(* Logix 5000 Rung export; software revision 20.05 *)

TYPE ILX34MBSCoilData :   // Coil Data
STRUCT
   Data : BOOL[576];
END_STRUCT
END_TYPE

TYPE ILX34MBSUTIL :
STRUCT
   Node : SINT;
   Function : SINT;
   NodeAddress : INT;
   Count : INT;
   ByteCount : SINT;
   IntAddress : INT;
   CountPlusIntAddr : INT;
   Swap : SINT;
   CmdTimer : TIMER[30];
   CurrentCmd : INT;
   CurrentCmdReset : BOOL;
   CmdDone : BOOL;
   TX_ASSY : SINT[82];
   TXID_Previous : SINT;
   RX_ASSY : SINT[90];
   RXID_Previous : SINT;
   RegBuffer : INT[72];
   CoilBuffer : ILX34MBSCoilData;
   MoveTo : INT;
   MoveFrom : INT;
   MasterTXQuery : BOOL;
   MasterRXResponse : BOOL;
   SlaveQuery : BOOL;
   WaitForResponse : BOOL;
   WaitTimer : TIMER;
   Error : SINT;
   WaitForError : BOOL;
   RegDataControl : CONTROL;
   InArraySize : INT;
   OutArraySize : INT;
   InputDiscreteArraySize : INT;
   OutputDiscreteArraySize : INT;
   InputRegisterArraySize : INT;
   OutputRegisterArraySize : INT;
   InputDiscreteArraySizem1 : INT;
   OutputDiscreteArraySizem1 : INT;
   InputRegisterArraySizem1 : INT;
   OutputRegisterArraySizem1 : INT;
   MaxDiscreteSize : INT;
   MaxRegisterSize : INT;
   Connection : BOOL;
END_STRUCT
END_TYPE

TYPE ILX34MBSData :   // Module Data Storage
STRUCT
   InputBit : BOOL[576];   // Coil/Input Input Data
   InputRegister : INT[500];   // Input/Holding Register Input Data
   OutputBit : BOOL[576];   // Coil/Input Output Data
   OutputRegister : INT[500];   // Input/Holding Register Output Data
END_STRUCT
END_TYPE

TYPE ILX34MBSCmd :   // Commands for module when used as a master.
STRUCT
   Enable : SINT;   // 0=Disable 1=Enable the command: Polling and Trigger allowed. 2=Enable the command: Trigger allowed only.
   Node : INT;   // Node address of the target device on the network (1-255).
   Function : SINT;   // Function code for the command. 1, 2, 3, 4, 5, 6, 15 and 16 allowed for master and slave. 8 allowed for slave only.
   DeviceAddress : DINT;   // Address in remote device associated with the command (0-65535).
   Count : INT;   // Number of points associated with the command.
   InternalAddress : DINT;
   PollInterval : DINT;   // Minimum number of milliseconds between issuance of command (0-2,147,483,647ms).
   Swap : SINT;
   Trigger : BOOL;   // 1=Trigger the message. Can be triggered any time command is enabled.
END_STRUCT
END_TYPE

TYPE ILX34MBSConfig :   // Configure the Module
STRUCT
   Type : SINT;   // 0=Master, 1=Slave
   Slave_ID : SINT;   // Slave ID (1-255)
   Baud_Rate : SINT;   // Baud Rate: 0=19200 2=2400 3=4800 4=9600 5=38400
   Serial_COM : SINT;   // 0=7N2 1=7E1 2=7O1 3=8N1 4=8N2 5=8E1 6=8O1
   Protocol : SINT;   // 0 = ASCII 1 = RTU
   RX_Length : SINT;   // Reserved
   TX_Length : SINT;   // Reserved
   Timeout : DINT;   // Timeout in centiseconds (1/100th of a second)
   Reserved01 : INT;   // Reserved
   Input_Status_Count_1X : INT;   // Input Status (1x) Maximum Address
   Reserved02 : INT;   // Reserved
   Output_Coil_Count_0X : INT;   // Output Coil (0x) Maximum Address
   Reserved03 : INT;   // Reserved
   Input_Register_Count_3X : INT;   // Input Register (3x) Maximum Address
   Reserved04 : INT;   // Reserved
   Holding_Register_Count_4X : INT;   // Holding Register (4x) Maximum Address
   Coldboot : BOOL;   // Reset Module to load configuration changes
END_STRUCT
END_TYPE

TYPE ILX34MBSStatus :   // Module Status
STRUCT
   Module : SINT;   // Module Status 1=Ready for Command 2=Processing Command 3=Waiting for Response 4=Processing Response
   RXCount : DINT;   // Number of messages received.
   TXCount : DINT;   // Number of messages transmitted.
   ErrorCount : DINT;   // Number of errors.
   CmdError : INT[30];
END_STRUCT
END_TYPE

TYPE ILX34MBSModuleDef :   // ILX34MBS Data Type
STRUCT
   DATA : ILX34MBSData;   // Data Storage
   STATUS : ILX34MBSStatus;   // Module Status
   MASTERCMD : ILX34MBSCmd[30];   // Master Commands
   UTIL : ILX34MBSUTIL;
END_STRUCT
END_TYPE

ADD_ON_INSTRUCTION AOI1734MBS_36   (* revision 1.10, vendor ProSoft Technology Inc., ExecutePrescan *)
// Add-On - L1y & 1734 Point I/O modules.
// Revision note:
// V1.7 - Resend command if stale
// V1.8 - Function Code 4 Swap for revision 1.15 or lower
// V1.9 - Built AOI in RSlogix v16
// V1.10 - Removed retranmission logic as it was causing addiitonal slave retransmissions.
// Help:
// Previous Version 1.8 was not able to open up in v16 Rslogix 5000.
// Built it back again to support v16 and up.
VAR_IN_OUT
   Connection_Input : SINT[90]; {required}
   Connection_Output : SINT[82]; {required}
   Connection_Config : INT[198]; {required}
        [5].0   // 0=Master 1=Slave
   MBS : ILX34MBSModuleDef; {required}
END_VAR
VAR
   ByteBuffer : SINT[72];
   ByteMoveBuffer : SINT[72];
   ByteSwappedRegister : INT[36];
   CurrentCmd : INT;
   CurrentSwapCount : INT;
   IntAddress : INT;
   MJFAULTS : DINT[12];
   ResetCommandTimer : TIMER;
   WordBuffer : INT[36];
   WordByteSwapBuffer : INT[36];
   WordByteSwapMoveBuffer : INT[36];
   WordMoveBuffer : INT[36];
   WordSwappedRegister : INT[36];
END_VAR

ROUTINE Logic   (* ladder *)
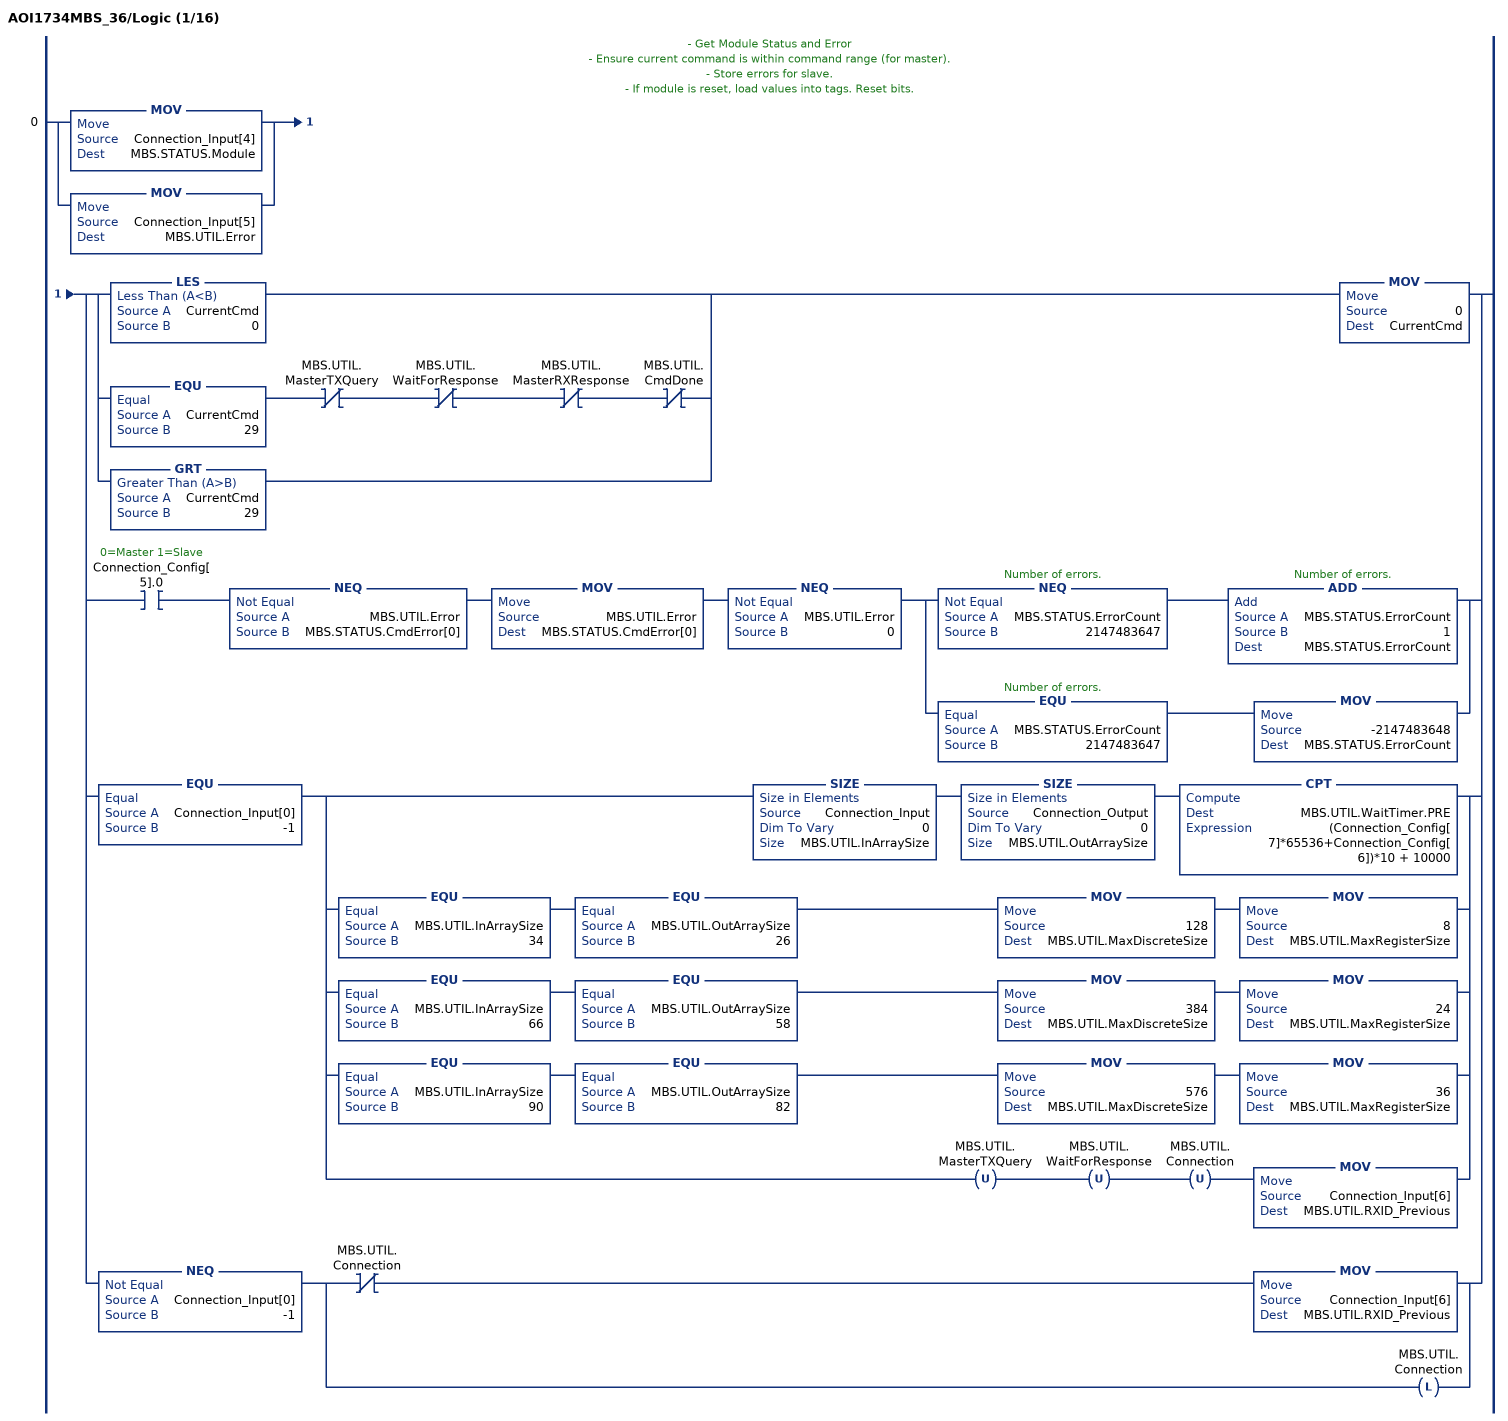
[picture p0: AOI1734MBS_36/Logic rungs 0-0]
   // - Get Module Status and Error
   // - Ensure current command is within command range (for master).
   // - Store errors for slave.
   // - If module is reset, load values into tags. Reset bits.
   0: [MOV(Connection_Input[4],MBS.STATUS.Module) ,MOV(Connection_Input[5],MBS.UTIL.Error) ][[LES(CurrentCmd,0) ,EQU(CurrentCmd,29) XIO(MBS.UTIL.MasterTXQuery) XIO(MBS.UTIL.WaitForResponse) XIO(MBS.UTIL.MasterRXResponse) XIO(MBS.UTIL.CmdDone) ,GRT(CurrentCmd,29) ] MOV(0,CurrentCmd) ,XIC(Connection_Config[5].0) NEQ(MBS.UTIL.Error,MBS.STATUS.CmdError[0]) MOV(MBS.UTIL.Error,MBS.STATUS.CmdError[0]) NEQ(MBS.UTIL.Error,0) [NEQ(MBS.STATUS.ErrorCount,2147483647) ADD(MBS.STATUS.ErrorCount,1,MBS.STATUS.ErrorCount) ,EQU(MBS.STATUS.ErrorCount,2147483647) MOV(-2147483648,MBS.STATUS.ErrorCount) ] ,EQU(Connection_Input[0],-1) [SIZE(Connection_Input,0,MBS.UTIL.InArraySize) SIZE(Connection_Output,0,MBS.UTIL.OutArraySize) CPT(MBS.UTIL.WaitTimer.PRE,(Connection_Config[7]*65536+Connection_Config[6])*10 + 10000) ,EQU(MBS.UTIL.InArraySize,34) EQU(MBS.UTIL.OutArraySize,26) MOV(128,MBS.UTIL.MaxDiscreteSize) MOV(8,MBS.UTIL.MaxRegisterSize) ,EQU(MBS.UTIL.InArraySize,66) EQU(MBS.UTIL.OutArraySize,58) MOV(384,MBS.UTIL.MaxDiscreteSize) MOV(24,MBS.UTIL.MaxRegisterSize) ,EQU(MBS.UTIL.InArraySize,90) EQU(MBS.UTIL.OutArraySize,82) MOV(576,MBS.UTIL.MaxDiscreteSize) MOV(36,MBS.UTIL.MaxRegisterSize) ,OTU(MBS.UTIL.MasterTXQuery) OTU(MBS.UTIL.WaitForResponse) OTU(MBS.UTIL.Connection) MOV(Connection_Input[6],MBS.UTIL.RXID_Previous) ] ,NEQ(Connection_Input[0],-1) [XIO(MBS.UTIL.Connection) MOV(Connection_Input[6],MBS.UTIL.RXID_Previous) ,OTL(MBS.UTIL.Connection) ] ];
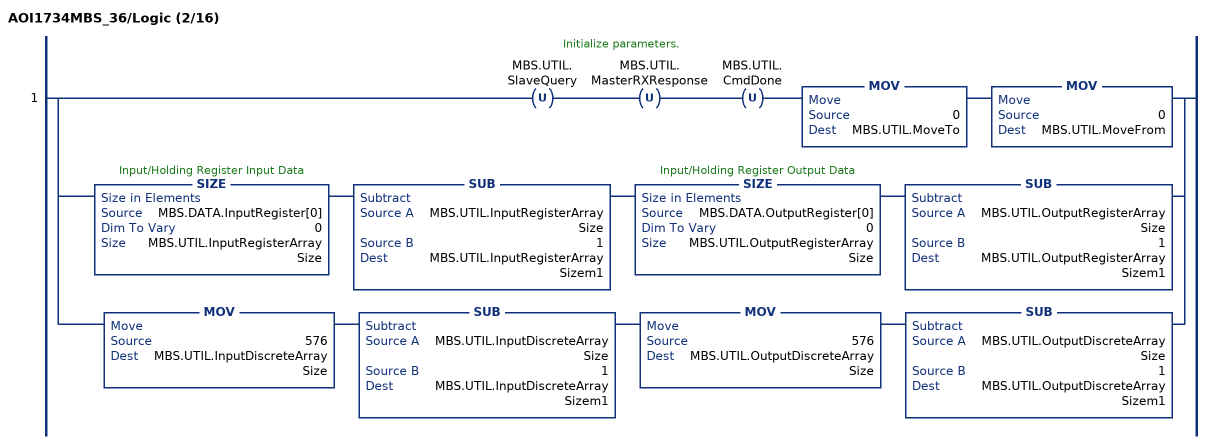
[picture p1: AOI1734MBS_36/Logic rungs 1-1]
   // Initialize parameters.
   1: [OTU(MBS.UTIL.SlaveQuery) OTU(MBS.UTIL.MasterRXResponse) OTU(MBS.UTIL.CmdDone) MOV(0,MBS.UTIL.MoveTo) MOV(0,MBS.UTIL.MoveFrom) ,SIZE(MBS.DATA.InputRegister[0],0,MBS.UTIL.InputRegisterArraySize) SUB(MBS.UTIL.InputRegisterArraySize,1,MBS.UTIL.InputRegisterArraySizem1) SIZE(MBS.DATA.OutputRegister[0],0,MBS.UTIL.OutputRegisterArraySize) SUB(MBS.UTIL.OutputRegisterArraySize,1,MBS.UTIL.OutputRegisterArraySizem1) ,MOV(576,MBS.UTIL.InputDiscreteArraySize) SUB(MBS.UTIL.InputDiscreteArraySize,1,MBS.UTIL.InputDiscreteArraySizem1) MOV(576,MBS.UTIL.OutputDiscreteArraySize) SUB(MBS.UTIL.OutputDiscreteArraySize,1,MBS.UTIL.OutputDiscreteArraySizem1) ];
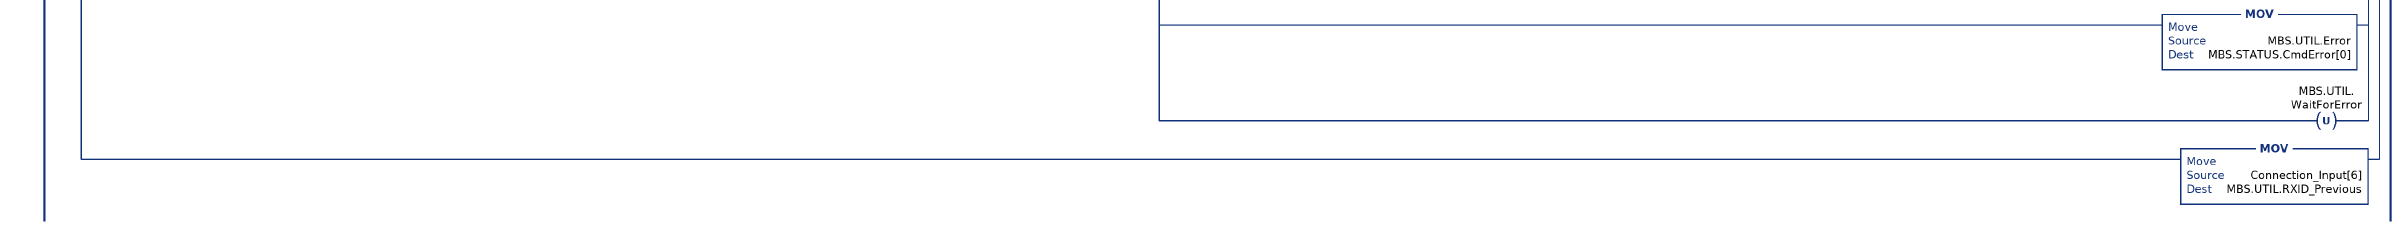
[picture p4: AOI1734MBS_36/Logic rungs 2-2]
   // Receive a message and store into buffer.
   // - If module is a master set response bit.
   // - If module is a slave set query bit (to set up response). Load query info into tags.
   // - If an error occurs in the slave, store type.
   2: NEQ(Connection_Input[6],MBS.UTIL.RXID_Previous)[XIO(Connection_Config[5].0) EQU(Connection_Input[4],1) ,XIC(Connection_Config[5].0) ]COP(Connection_Input[0],MBS.UTIL.RX_ASSY[0],MBS.UTIL.InArraySize)[[MOV(MBS.UTIL.RX_ASSY[4],MBS.STATUS.Module) ,MOV(MBS.UTIL.RX_ASSY[5],MBS.UTIL.Error) ] ,EQU(MBS.UTIL.Error,0) [NEQ(MBS.STATUS.RXCount,2147483647) ADD(1,MBS.STATUS.RXCount,MBS.STATUS.RXCount) ,EQU(MBS.STATUS.RXCount,2147483647) MOV(-2147483648,MBS.STATUS.RXCount) ] ,EQU(MBS.UTIL.Error,0) [XIO(Connection_Config[5].0) EQU(MBS.UTIL.RX_ASSY[8],MBS.UTIL.Function) OTL(MBS.UTIL.MasterRXResponse) ,XIC(Connection_Config[5].0) NEQ(MBS.UTIL.RX_ASSY[8],8) [MOV(MBS.UTIL.RX_ASSY[7],MBS.UTIL.Node) MOV(MBS.UTIL.RX_ASSY[8],MBS.UTIL.Function) COP(MBS.UTIL.RX_ASSY[9],MBS.UTIL.NodeAddress,1) COP(MBS.UTIL.RX_ASSY[11],MBS.UTIL.Count,1) COP(MBS.UTIL.RX_ASSY[9],MBS.UTIL.IntAddress,1) ADD(MBS.UTIL.Count,MBS.UTIL.IntAddress,MBS.UTIL.CountPlusIntAddr) ,[[LIM(1,MBS.UTIL.Function,2) [EQU(MBS.UTIL.Function,1) SUB(MBS.UTIL.IntAddress,Connection_Config[9],MBS.UTIL.IntAddress) ,EQU(MBS.UTIL.Function,2) SUB(MBS.UTIL.IntAddress,Connection_Config[11],MBS.UTIL.IntAddress) ] LIM(0,MBS.UTIL.IntAddress,MBS.UTIL.OutputDiscreteArraySizem1) LIM(1,MBS.UTIL.CountPlusIntAddr,MBS.UTIL.OutputDiscreteArraySize) ,EQU(MBS.UTIL.Function,15) SUB(MBS.UTIL.IntAddress,Connection_Config[9],MBS.UTIL.IntAddress) LIM(0,MBS.UTIL.IntAddress,MBS.UTIL.InputDiscreteArraySizem1) LIM(1,MBS.UTIL.CountPlusIntAddr,MBS.UTIL.InputDiscreteArraySize) ] LIM(1,MBS.UTIL.Count,MBS.UTIL.MaxDiscreteSize) ,[LIM(3,MBS.UTIL.Function,4) [EQU(MBS.UTIL.Function,3) SUB(MBS.UTIL.IntAddress,Connection_Config[15],MBS.UTIL.IntAddress) ,EQU(MBS.UTIL.Function,4) SUB(MBS.UTIL.IntAddress,Connection_Config[13],MBS.UTIL.IntAddress) ] LIM(0,MBS.UTIL.IntAddress,MBS.UTIL.OutputRegisterArraySizem1) LIM(1,MBS.UTIL.CountPlusIntAddr,MBS.UTIL.OutputRegisterArraySize) ,EQU(MBS.UTIL.Function,16) SUB(MBS.UTIL.IntAddress,Connection_Config[15],MBS.UTIL.IntAddress) LIM(0,MBS.UTIL.IntAddress,MBS.UTIL.InputRegisterArraySizem1) LIM(1,MBS.UTIL.CountPlusIntAddr,MBS.UTIL.InputRegisterArraySize) ] LIM(1,MBS.UTIL.Count,MBS.UTIL.MaxRegisterSize) ,EQU(MBS.UTIL.Function,5) LIM(0,MBS.UTIL.IntAddress,MBS.UTIL.InputDiscreteArraySizem1) ,EQU(MBS.UTIL.Function,6) SUB(MBS.UTIL.IntAddress,Connection_Config[15],MBS.UTIL.IntAddress) LIM(0,MBS.UTIL.IntAddress,MBS.UTIL.InputRegisterArraySizem1) ] [OTL(MBS.UTIL.SlaveQuery) ,MOV(MBS.UTIL.IntAddress,IntAddress) ] ] ] ,XIC(Connection_Config[5].0) NEQ(MBS.UTIL.Error,1) NEQ(MBS.UTIL.Error,2) NEQ(MBS.UTIL.Error,3) MOV(MBS.UTIL.Error,MBS.STATUS.CmdError[0]) NEQ(MBS.UTIL.Error,0) [NEQ(MBS.STATUS.ErrorCount,2147483647) ADD(MBS.STATUS.ErrorCount,1,MBS.STATUS.ErrorCount) ,EQU(MBS.STATUS.ErrorCount,2147483647) MOV(-2147483648,MBS.STATUS.ErrorCount) ,MOV(MBS.UTIL.Error,MBS.STATUS.CmdError[0]) ,OTU(MBS.UTIL.WaitForError) ] ,MOV(Connection_Input[6],MBS.UTIL.RXID_Previous) ];
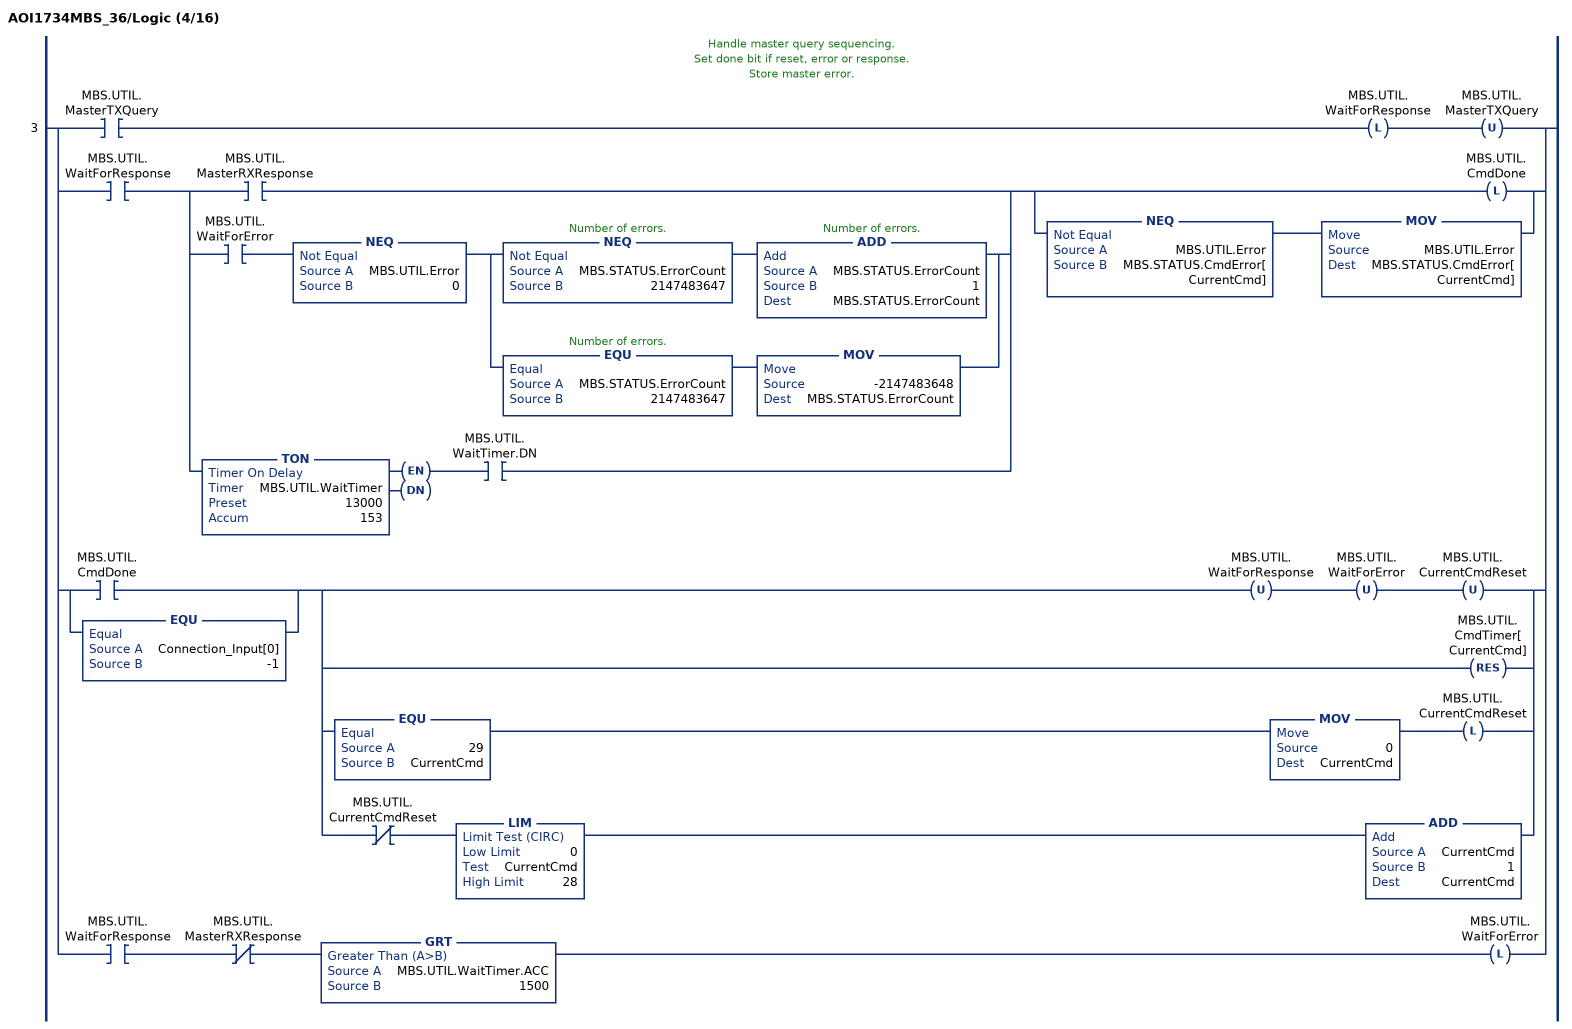
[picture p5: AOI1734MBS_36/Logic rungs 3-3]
   // Handle master query sequencing.
   // Set done bit if reset, error or response.
   // Store master error.
   3: [XIC(MBS.UTIL.MasterTXQuery) OTL(MBS.UTIL.WaitForResponse) OTU(MBS.UTIL.MasterTXQuery) ,XIC(MBS.UTIL.WaitForResponse) [XIC(MBS.UTIL.MasterRXResponse) ,XIC(MBS.UTIL.WaitForError) NEQ(MBS.UTIL.Error,0) [NEQ(MBS.STATUS.ErrorCount,2147483647) ADD(MBS.STATUS.ErrorCount,1,MBS.STATUS.ErrorCount) ,EQU(MBS.STATUS.ErrorCount,2147483647) MOV(-2147483648,MBS.STATUS.ErrorCount) ] ,TON(MBS.UTIL.WaitTimer,13000,153) XIC(MBS.UTIL.WaitTimer.DN) ] [OTL(MBS.UTIL.CmdDone) ,NEQ(MBS.UTIL.Error,MBS.STATUS.CmdError[CurrentCmd]) MOV(MBS.UTIL.Error,MBS.STATUS.CmdError[CurrentCmd]) ] ,[XIC(MBS.UTIL.CmdDone) ,EQU(Connection_Input[0],-1) ] [OTU(MBS.UTIL.WaitForResponse) OTU(MBS.UTIL.WaitForError) OTU(MBS.UTIL.CurrentCmdReset) ,RES(MBS.UTIL.CmdTimer[CurrentCmd]) ,EQU(29,CurrentCmd) MOV(0,CurrentCmd) OTL(MBS.UTIL.CurrentCmdReset) ,XIO(MBS.UTIL.CurrentCmdReset) LIM(0,CurrentCmd,28) ADD(CurrentCmd,1,CurrentCmd) ] ,XIC(MBS.UTIL.WaitForResponse) XIO(MBS.UTIL.MasterRXResponse) GRT(MBS.UTIL.WaitTimer.ACC,1500) OTL(MBS.UTIL.WaitForError) ];
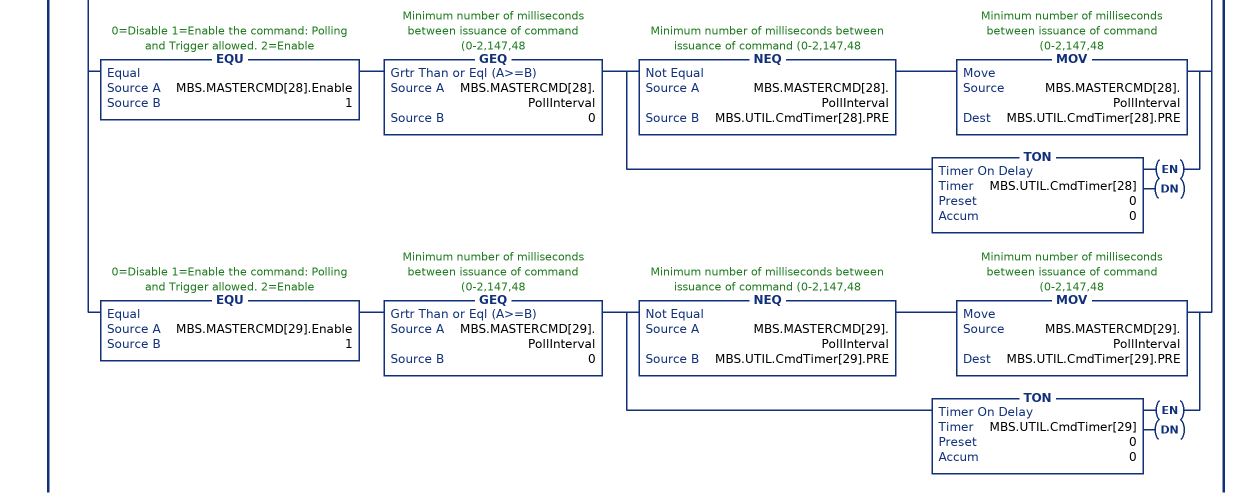
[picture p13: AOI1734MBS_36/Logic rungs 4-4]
   // Master command timers (from Poll Interval).
   // A timer runs only when command enabled = 1. Timers are reset in rung above.
   4: XIO(Connection_Config[5].0)[EQU(MBS.MASTERCMD[0].Enable,1) GEQ(MBS.MASTERCMD[0].PollInterval,0) [NEQ(MBS.MASTERCMD[0].PollInterval,MBS.UTIL.CmdTimer[0].PRE) MOV(MBS.MASTERCMD[0].PollInterval,MBS.UTIL.CmdTimer[0].PRE) ,TON(MBS.UTIL.CmdTimer[0],0,0) ] ,EQU(MBS.MASTERCMD[1].Enable,1) GEQ(MBS.MASTERCMD[1].PollInterval,0) [NEQ(MBS.MASTERCMD[1].PollInterval,MBS.UTIL.CmdTimer[1].PRE) MOV(MBS.MASTERCMD[1].PollInterval,MBS.UTIL.CmdTimer[1].PRE) ,TON(MBS.UTIL.CmdTimer[1],0,0) ] ,EQU(MBS.MASTERCMD[2].Enable,1) GEQ(MBS.MASTERCMD[2].PollInterval,0) [NEQ(MBS.MASTERCMD[2].PollInterval,MBS.UTIL.CmdTimer[2].PRE) MOV(MBS.MASTERCMD[2].PollInterval,MBS.UTIL.CmdTimer[2].PRE) ,TON(MBS.UTIL.CmdTimer[2],0,0) ] ,EQU(MBS.MASTERCMD[3].Enable,1) GEQ(MBS.MASTERCMD[3].PollInterval,0) [NEQ(MBS.MASTERCMD[3].PollInterval,MBS.UTIL.CmdTimer[3].PRE) MOV(MBS.MASTERCMD[3].PollInterval,MBS.UTIL.CmdTimer[3].PRE) ,TON(MBS.UTIL.CmdTimer[3],0,0) ] ,EQU(MBS.MASTERCMD[4].Enable,1) GEQ(MBS.MASTERCMD[4].PollInterval,0) [NEQ(MBS.MASTERCMD[4].PollInterval,MBS.UTIL.CmdTimer[4].PRE) MOV(MBS.MASTERCMD[4].PollInterval,MBS.UTIL.CmdTimer[4].PRE) ,TON(MBS.UTIL.CmdTimer[4],0,0) ] ,EQU(MBS.MASTERCMD[5].Enable,1) GEQ(MBS.MASTERCMD[5].PollInterval,0) [NEQ(MBS.MASTERCMD[5].PollInterval,MBS.UTIL.CmdTimer[5].PRE) MOV(MBS.MASTERCMD[5].PollInterval,MBS.UTIL.CmdTimer[5].PRE) ,TON(MBS.UTIL.CmdTimer[5],0,3) ] ,EQU(MBS.MASTERCMD[6].Enable,1) GEQ(MBS.MASTERCMD[6].PollInterval,0) [NEQ(MBS.MASTERCMD[6].PollInterval,MBS.UTIL.CmdTimer[6].PRE) MOV(MBS.MASTERCMD[6].PollInterval,MBS.UTIL.CmdTimer[6].PRE) ,TON(MBS.UTIL.CmdTimer[6],0,4) ] ,EQU(MBS.MASTERCMD[7].Enable,1) GEQ(MBS.MASTERCMD[7].PollInterval,0) [NEQ(MBS.MASTERCMD[7].PollInterval,MBS.UTIL.CmdTimer[7].PRE) MOV(MBS.MASTERCMD[7].PollInterval,MBS.UTIL.CmdTimer[7].PRE) ,TON(MBS.UTIL.CmdTimer[7],0,0) ] ,EQU(MBS.MASTERCMD[8].Enable,1) GEQ(MBS.MASTERCMD[8].PollInterval,0) [NEQ(MBS.MASTERCMD[8].PollInterval,MBS.UTIL.CmdTimer[8].PRE) MOV(MBS.MASTERCMD[8].PollInterval,MBS.UTIL.CmdTimer[8].PRE) ,TON(MBS.UTIL.CmdTimer[8],0,0) ] ,EQU(MBS.MASTERCMD[9].Enable,1) GEQ(MBS.MASTERCMD[9].PollInterval,0) [NEQ(MBS.MASTERCMD[9].PollInterval,MBS.UTIL.CmdTimer[9].PRE) MOV(MBS.MASTERCMD[9].PollInterval,MBS.UTIL.CmdTimer[9].PRE) ,TON(MBS.UTIL.CmdTimer[9],0,0) ] ,EQU(MBS.MASTERCMD[10].Enable,1) GEQ(MBS.MASTERCMD[10].PollInterval,0) [NEQ(MBS.MASTERCMD[10].PollInterval,MBS.UTIL.CmdTimer[10].PRE) MOV(MBS.MASTERCMD[10].PollInterval,MBS.UTIL.CmdTimer[10].PRE) ,TON(MBS.UTIL.CmdTimer[10],0,0) ] ,EQU(MBS.MASTERCMD[11].Enable,1) GEQ(MBS.MASTERCMD[11].PollInterval,0) [NEQ(MBS.MASTERCMD[11].PollInterval,MBS.UTIL.CmdTimer[11].PRE) MOV(MBS.MASTERCMD[11].PollInterval,MBS.UTIL.CmdTimer[11].PRE) ,TON(MBS.UTIL.CmdTimer[11],0,0) ] ,EQU(MBS.MASTERCMD[12].Enable,1) GEQ(MBS.MASTERCMD[12].PollInterval,0) [NEQ(MBS.MASTERCMD[12].PollInterval,MBS.UTIL.CmdTimer[12].PRE) MOV(MBS.MASTERCMD[12].PollInterval,MBS.UTIL.CmdTimer[12].PRE) ,TON(MBS.UTIL.CmdTimer[12],0,0) ] ,EQU(MBS.MASTERCMD[13].Enable,1) GEQ(MBS.MASTERCMD[13].PollInterval,0) [NEQ(MBS.MASTERCMD[13].PollInterval,MBS.UTIL.CmdTimer[13].PRE) MOV(MBS.MASTERCMD[13].PollInterval,MBS.UTIL.CmdTimer[13].PRE) ,TON(MBS.UTIL.CmdTimer[13],0,0) ] ,EQU(MBS.MASTERCMD[14].Enable,1) GEQ(MBS.MASTERCMD[14].PollInterval,0) [NEQ(MBS.MASTERCMD[14].PollInterval,MBS.UTIL.CmdTimer[14].PRE) MOV(MBS.MASTERCMD[14].PollInterval,MBS.UTIL.CmdTimer[14].PRE) ,TON(MBS.UTIL.CmdTimer[14],0,0) ] ,EQU(MBS.MASTERCMD[15].Enable,1) GEQ(MBS.MASTERCMD[15].PollInterval,0) [NEQ(MBS.MASTERCMD[15].PollInterval,MBS.UTIL.CmdTimer[15].PRE) MOV(MBS.MASTERCMD[15].PollInterval,MBS.UTIL.CmdTimer[15].PRE) ,TON(MBS.UTIL.CmdTimer[15],0,0) ] ,EQU(MBS.MASTERCMD[16].Enable,1) GEQ(MBS.MASTERCMD[16].PollInterval,0) [NEQ(MBS.MASTERCMD[16].PollInterval,MBS.UTIL.CmdTimer[16].PRE) MOV(MBS.MASTERCMD[16].PollInterval,MBS.UTIL.CmdTimer[16].PRE) ,TON(MBS.UTIL.CmdTimer[16],0,0) ] ,EQU(MBS.MASTERCMD[17].Enable,1) GEQ(MBS.MASTERCMD[17].PollInterval,0) [NEQ(MBS.MASTERCMD[17].PollInterval,MBS.UTIL.CmdTimer[17].PRE) MOV(MBS.MASTERCMD[17].PollInterval,MBS.UTIL.CmdTimer[17].PRE) ,TON(MBS.UTIL.CmdTimer[17],0,0) ] ,EQU(MBS.MASTERCMD[18].Enable,1) GEQ(MBS.MASTERCMD[18].PollInterval,0) [NEQ(MBS.MASTERCMD[18].PollInterval,MBS.UTIL.CmdTimer[18].PRE) MOV(MBS.MASTERCMD[18].PollInterval,MBS.UTIL.CmdTimer[18].PRE) ,TON(MBS.UTIL.CmdTimer[18],2000,0) ] ,EQU(MBS.MASTERCMD[19].Enable,1) GEQ(MBS.MASTERCMD[19].PollInterval,0) [NEQ(MBS.MASTERCMD[19].PollInterval,MBS.UTIL.CmdTimer[19].PRE) MOV(MBS.MASTERCMD[19].PollInterval,MBS.UTIL.CmdTimer[19].PRE) ,TON(MBS.UTIL.CmdTimer[19],0,0) ] ,EQU(MBS.MASTERCMD[20].Enable,1) GEQ(MBS.MASTERCMD[20].PollInterval,0) [NEQ(MBS.MASTERCMD[20].PollInterval,MBS.UTIL.CmdTimer[20].PRE) MOV(MBS.MASTERCMD[20].PollInterval,MBS.UTIL.CmdTimer[20].PRE) ,TON(MBS.UTIL.CmdTimer[20],0,0) ] ,EQU(MBS.MASTERCMD[21].Enable,1) GEQ(MBS.MASTERCMD[21].PollInterval,0) [NEQ(MBS.MASTERCMD[21].PollInterval,MBS.UTIL.CmdTimer[21].PRE) MOV(MBS.MASTERCMD[21].PollInterval,MBS.UTIL.CmdTimer[21].PRE) ,TON(MBS.UTIL.CmdTimer[21],0,0) ] ,EQU(MBS.MASTERCMD[22].Enable,1) GEQ(MBS.MASTERCMD[22].PollInterval,0) [NEQ(MBS.MASTERCMD[22].PollInterval,MBS.UTIL.CmdTimer[22].PRE) MOV(MBS.MASTERCMD[22].PollInterval,MBS.UTIL.CmdTimer[22].PRE) ,TON(MBS.UTIL.CmdTimer[22],0,0) ] ,EQU(MBS.MASTERCMD[23].Enable,1) GEQ(MBS.MASTERCMD[23].PollInterval,0) [NEQ(MBS.MASTERCMD[23].PollInterval,MBS.UTIL.CmdTimer[23].PRE) MOV(MBS.MASTERCMD[23].PollInterval,MBS.UTIL.CmdTimer[23].PRE) ,TON(MBS.UTIL.CmdTimer[23],0,0) ] ,EQU(MBS.MASTERCMD[24].Enable,1) GEQ(MBS.MASTERCMD[24].PollInterval,0) [NEQ(MBS.MASTERCMD[24].PollInterval,MBS.UTIL.CmdTimer[24].PRE) MOV(MBS.MASTERCMD[24].PollInterval,MBS.UTIL.CmdTimer[24].PRE) ,TON(MBS.UTIL.CmdTimer[24],0,0) ] ,EQU(MBS.MASTERCMD[25].Enable,1) GEQ(MBS.MASTERCMD[25].PollInterval,0) [NEQ(MBS.MASTERCMD[25].PollInterval,MBS.UTIL.CmdTimer[25].PRE) MOV(MBS.MASTERCMD[25].PollInterval,MBS.UTIL.CmdTimer[25].PRE) ,TON(MBS.UTIL.CmdTimer[25],0,0) ] ,EQU(MBS.MASTERCMD[26].Enable,1) GEQ(MBS.MASTERCMD[26].PollInterval,0) [NEQ(MBS.MASTERCMD[26].PollInterval,MBS.UTIL.CmdTimer[26].PRE) MOV(MBS.MASTERCMD[26].PollInterval,MBS.UTIL.CmdTimer[26].PRE) ,TON(MBS.UTIL.CmdTimer[26],0,0) ] ,EQU(MBS.MASTERCMD[27].Enable,1) GEQ(MBS.MASTERCMD[27].PollInterval,0) [NEQ(MBS.MASTERCMD[27].PollInterval,MBS.UTIL.CmdTimer[27].PRE) MOV(MBS.MASTERCMD[27].PollInterval,MBS.UTIL.CmdTimer[27].PRE) ,TON(MBS.UTIL.CmdTimer[27],0,0) ] ,EQU(MBS.MASTERCMD[28].Enable,1) GEQ(MBS.MASTERCMD[28].PollInterval,0) [NEQ(MBS.MASTERCMD[28].PollInterval,MBS.UTIL.CmdTimer[28].PRE) MOV(MBS.MASTERCMD[28].PollInterval,MBS.UTIL.CmdTimer[28].PRE) ,TON(MBS.UTIL.CmdTimer[28],0,0) ] ,EQU(MBS.MASTERCMD[29].Enable,1) GEQ(MBS.MASTERCMD[29].PollInterval,0) [NEQ(MBS.MASTERCMD[29].PollInterval,MBS.UTIL.CmdTimer[29].PRE) MOV(MBS.MASTERCMD[29].PollInterval,MBS.UTIL.CmdTimer[29].PRE) ,TON(MBS.UTIL.CmdTimer[29],0,0) ] ];
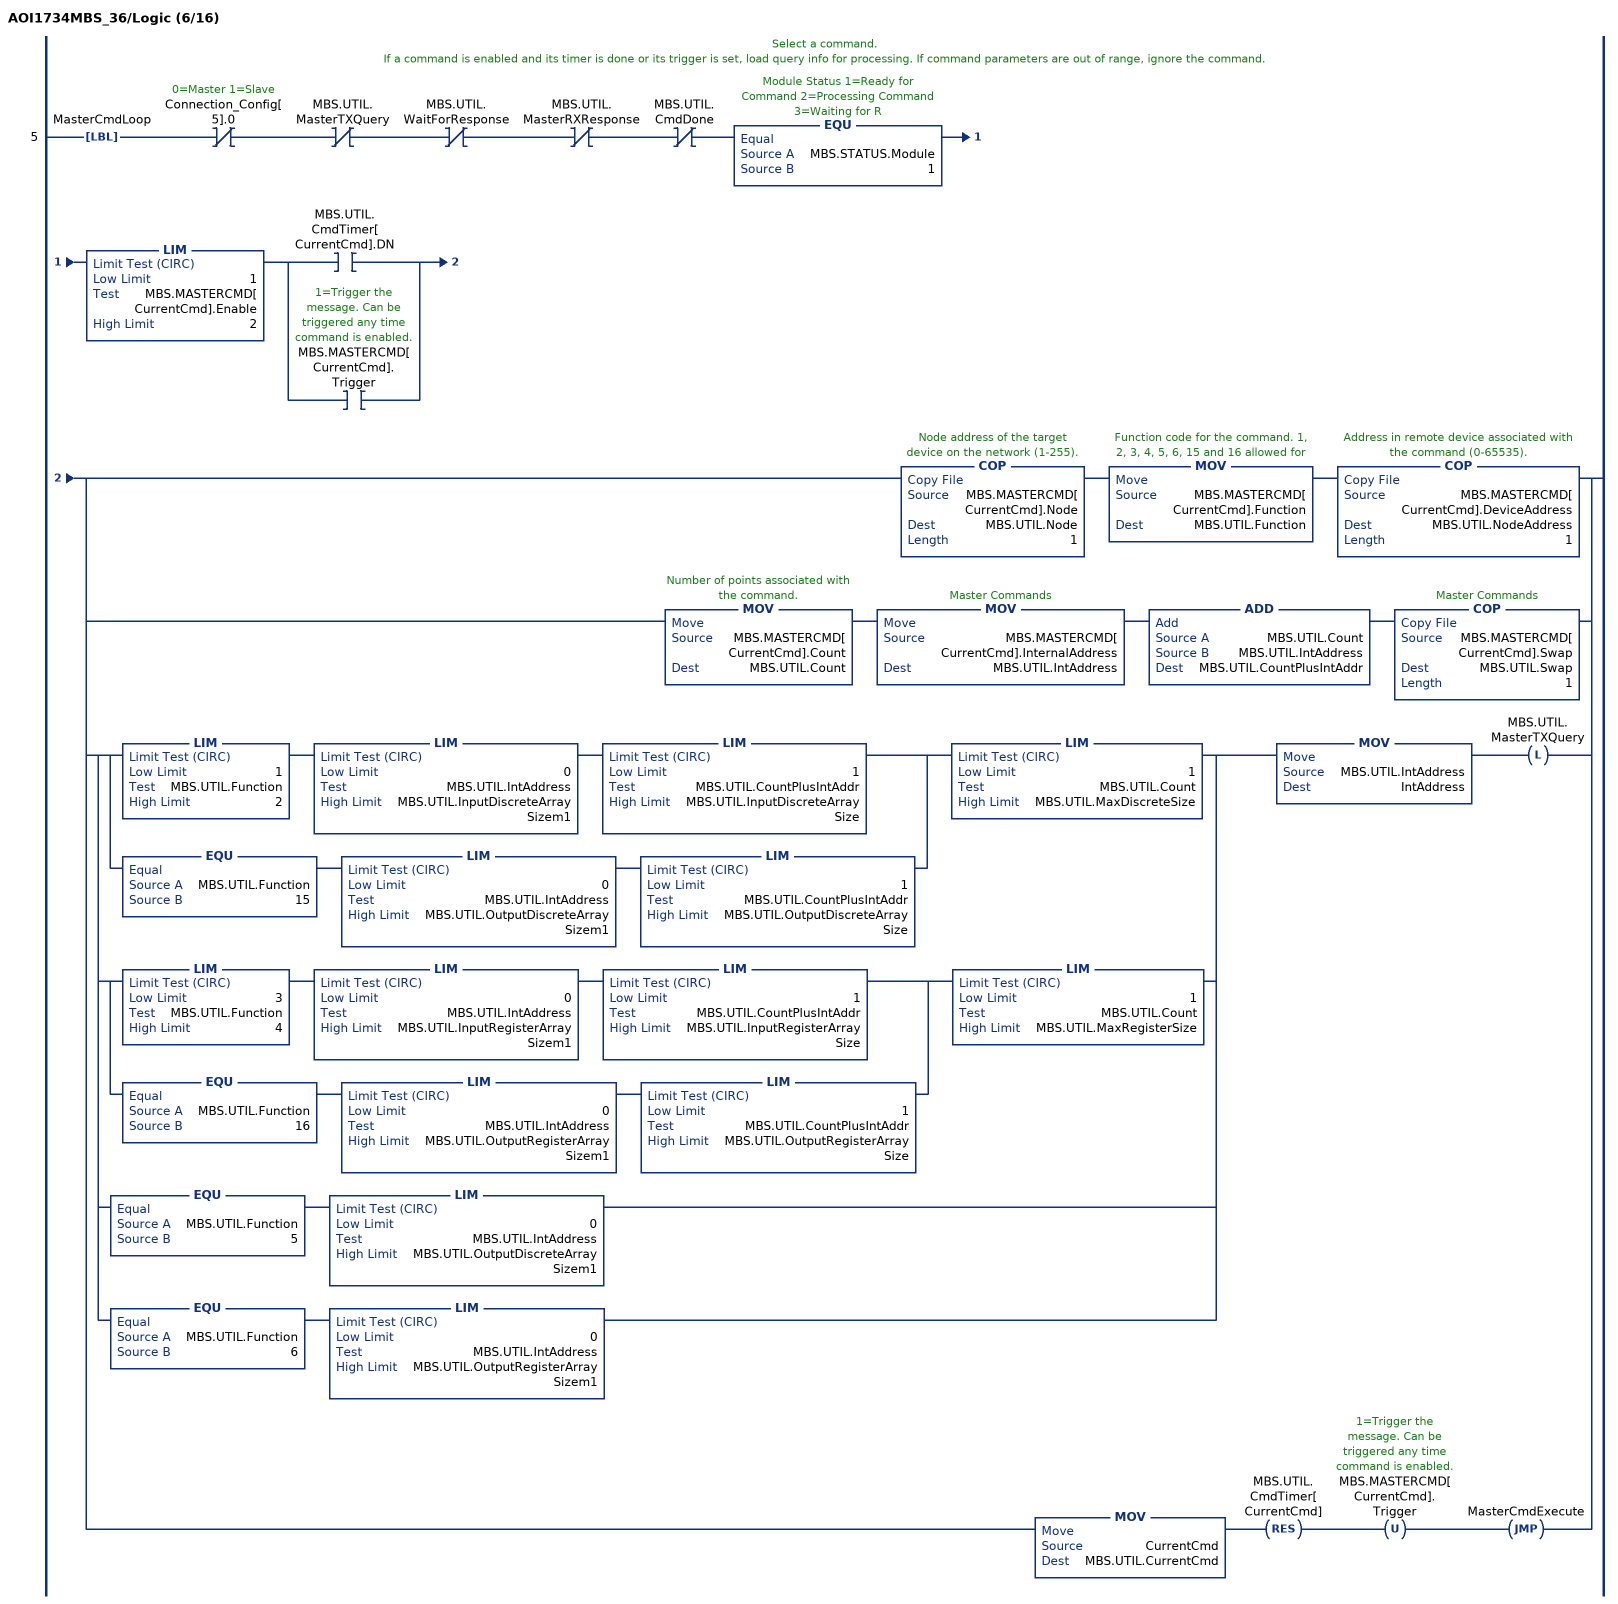
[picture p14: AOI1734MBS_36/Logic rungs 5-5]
   // Select a command.
   // If a command is enabled and its timer is done or its trigger is set, load query info for processing. If command parameters are out of range, ignore the command.
   5: LBL(MasterCmdLoop)XIO(Connection_Config[5].0)XIO(MBS.UTIL.MasterTXQuery)XIO(MBS.UTIL.WaitForResponse)XIO(MBS.UTIL.MasterRXResponse)XIO(MBS.UTIL.CmdDone)EQU(MBS.STATUS.Module,1)LIM(1,MBS.MASTERCMD[CurrentCmd].Enable,2)[XIC(MBS.UTIL.CmdTimer[CurrentCmd].DN) ,XIC(MBS.MASTERCMD[CurrentCmd].Trigger) ][[COP(MBS.MASTERCMD[CurrentCmd].Node,MBS.UTIL.Node,1) MOV(MBS.MASTERCMD[CurrentCmd].Function,MBS.UTIL.Function) COP(MBS.MASTERCMD[CurrentCmd].DeviceAddress,MBS.UTIL.NodeAddress,1) ,MOV(MBS.MASTERCMD[CurrentCmd].Count,MBS.UTIL.Count) MOV(MBS.MASTERCMD[CurrentCmd].InternalAddress,MBS.UTIL.IntAddress) ADD(MBS.UTIL.Count,MBS.UTIL.IntAddress,MBS.UTIL.CountPlusIntAddr) COP(MBS.MASTERCMD[CurrentCmd].Swap,MBS.UTIL.Swap,1) ] ,[[LIM(1,MBS.UTIL.Function,2) LIM(0,MBS.UTIL.IntAddress,MBS.UTIL.InputDiscreteArraySizem1) LIM(1,MBS.UTIL.CountPlusIntAddr,MBS.UTIL.InputDiscreteArraySize) ,EQU(MBS.UTIL.Function,15) LIM(0,MBS.UTIL.IntAddress,MBS.UTIL.OutputDiscreteArraySizem1) LIM(1,MBS.UTIL.CountPlusIntAddr,MBS.UTIL.OutputDiscreteArraySize) ] LIM(1,MBS.UTIL.Count,MBS.UTIL.MaxDiscreteSize) ,[LIM(3,MBS.UTIL.Function,4) LIM(0,MBS.UTIL.IntAddress,MBS.UTIL.InputRegisterArraySizem1) LIM(1,MBS.UTIL.CountPlusIntAddr,MBS.UTIL.InputRegisterArraySize) ,EQU(MBS.UTIL.Function,16) LIM(0,MBS.UTIL.IntAddress,MBS.UTIL.OutputRegisterArraySizem1) LIM(1,MBS.UTIL.CountPlusIntAddr,MBS.UTIL.OutputRegisterArraySize) ] LIM(1,MBS.UTIL.Count,MBS.UTIL.MaxRegisterSize) ,EQU(MBS.UTIL.Function,5) LIM(0,MBS.UTIL.IntAddress,MBS.UTIL.OutputDiscreteArraySizem1) ,EQU(MBS.UTIL.Function,6) LIM(0,MBS.UTIL.IntAddress,MBS.UTIL.OutputRegisterArraySizem1) ] MOV(MBS.UTIL.IntAddress,IntAddress) OTL(MBS.UTIL.MasterTXQuery) ,MOV(CurrentCmd,MBS.UTIL.CurrentCmd) RES(MBS.UTIL.CmdTimer[CurrentCmd]) OTU(MBS.MASTERCMD[CurrentCmd].Trigger) JMP(MasterCmdExecute) ];
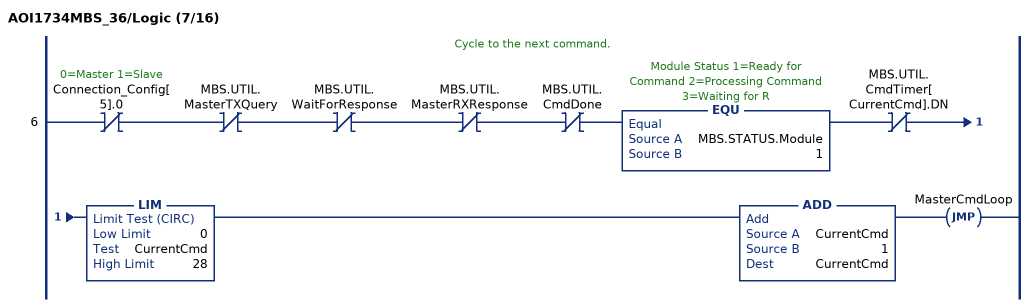
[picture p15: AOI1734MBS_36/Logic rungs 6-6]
   // Cycle to the next command.
   6: XIO(Connection_Config[5].0)XIO(MBS.UTIL.MasterTXQuery)XIO(MBS.UTIL.WaitForResponse)XIO(MBS.UTIL.MasterRXResponse)XIO(MBS.UTIL.CmdDone)EQU(MBS.STATUS.Module,1)XIO(MBS.UTIL.CmdTimer[CurrentCmd].DN)LIM(0,CurrentCmd,28)ADD(CurrentCmd,1,CurrentCmd)JMP(MasterCmdLoop);
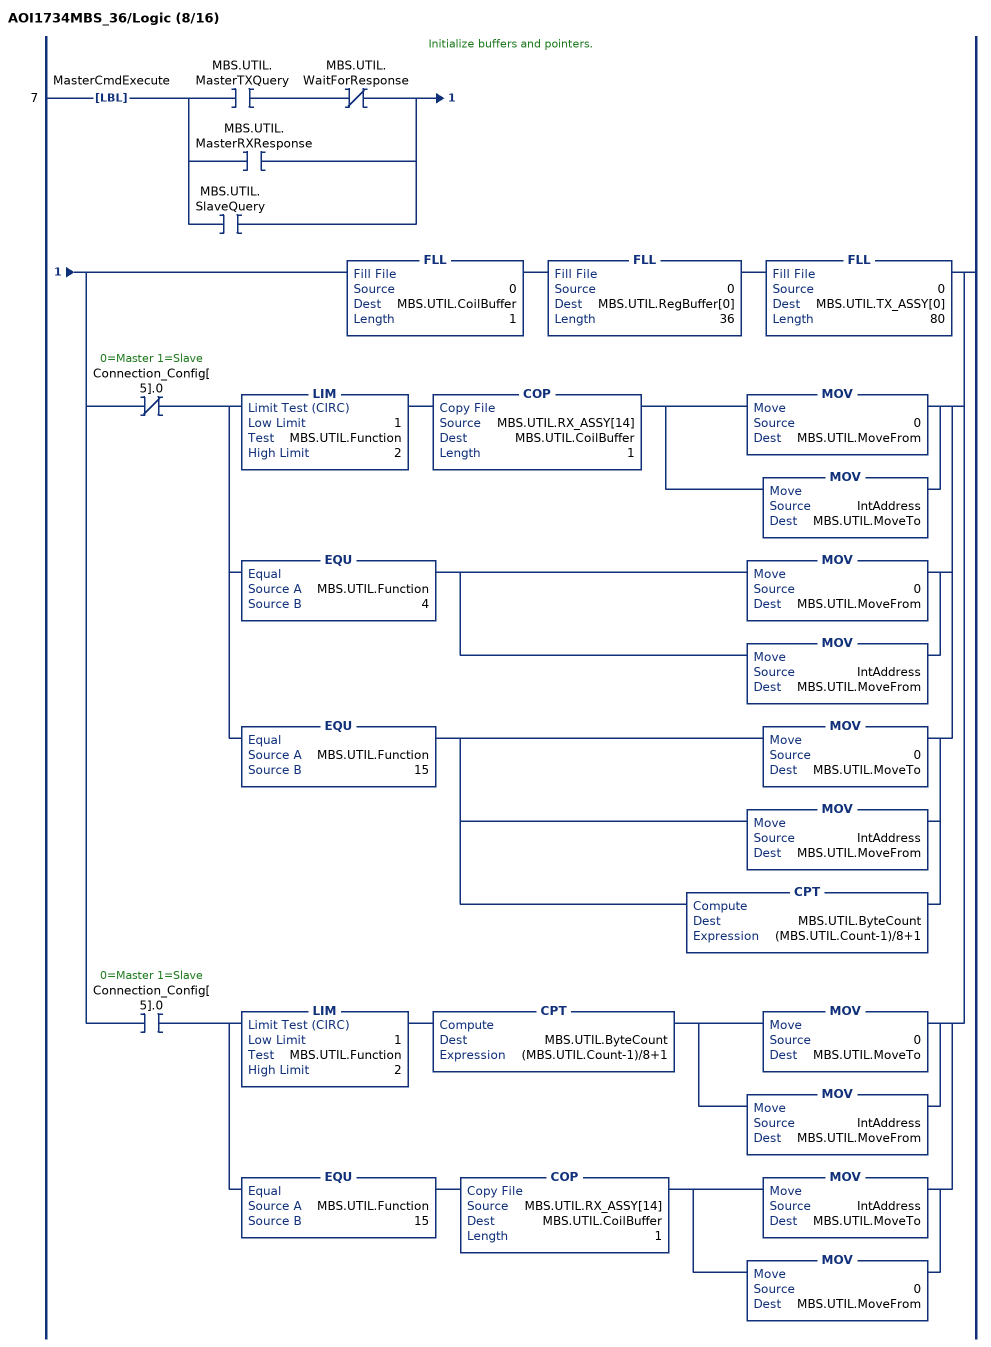
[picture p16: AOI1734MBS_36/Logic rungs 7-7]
   // Initialize buffers and pointers.
   7: LBL(MasterCmdExecute)[XIC(MBS.UTIL.MasterTXQuery) XIO(MBS.UTIL.WaitForResponse) ,XIC(MBS.UTIL.MasterRXResponse) ,XIC(MBS.UTIL.SlaveQuery) ][FLL(0,MBS.UTIL.CoilBuffer,1) FLL(0,MBS.UTIL.RegBuffer[0],36) FLL(0,MBS.UTIL.TX_ASSY[0],80) ,XIO(Connection_Config[5].0) [LIM(1,MBS.UTIL.Function,2) COP(MBS.UTIL.RX_ASSY[14],MBS.UTIL.CoilBuffer,1) [MOV(0,MBS.UTIL.MoveFrom) ,MOV(IntAddress,MBS.UTIL.MoveTo) ] ,EQU(MBS.UTIL.Function,4) [MOV(0,MBS.UTIL.MoveFrom) ,MOV(IntAddress,MBS.UTIL.MoveFrom) ] ,EQU(MBS.UTIL.Function,15) [MOV(0,MBS.UTIL.MoveTo) ,MOV(IntAddress,MBS.UTIL.MoveFrom) ,CPT(MBS.UTIL.ByteCount,(MBS.UTIL.Count-1)/8+1) ] ] ,XIC(Connection_Config[5].0) [LIM(1,MBS.UTIL.Function,2) CPT(MBS.UTIL.ByteCount,(MBS.UTIL.Count-1)/8+1) [MOV(0,MBS.UTIL.MoveTo) ,MOV(IntAddress,MBS.UTIL.MoveFrom) ] ,EQU(MBS.UTIL.Function,15) COP(MBS.UTIL.RX_ASSY[14],MBS.UTIL.CoilBuffer,1) [MOV(IntAddress,MBS.UTIL.MoveTo) ,MOV(0,MBS.UTIL.MoveFrom) ] ] ];
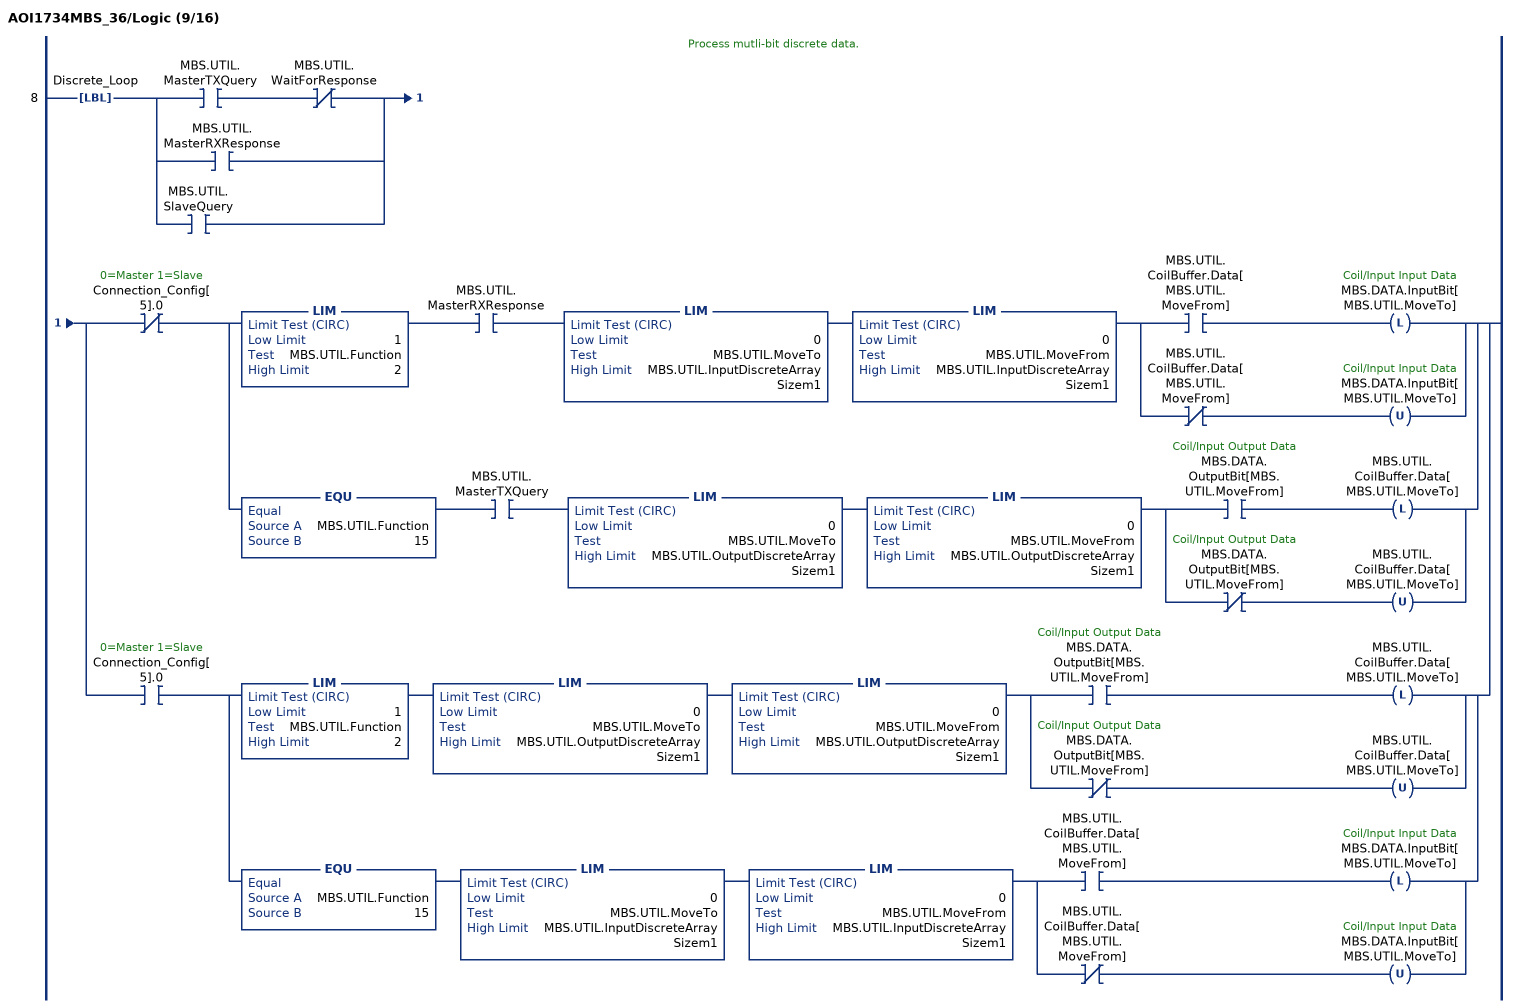
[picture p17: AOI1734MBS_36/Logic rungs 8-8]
   // Process mutli-bit discrete data.
   8: LBL(Discrete_Loop)[XIC(MBS.UTIL.MasterTXQuery) XIO(MBS.UTIL.WaitForResponse) ,XIC(MBS.UTIL.MasterRXResponse) ,XIC(MBS.UTIL.SlaveQuery) ][XIO(Connection_Config[5].0) [LIM(1,MBS.UTIL.Function,2) XIC(MBS.UTIL.MasterRXResponse) LIM(0,MBS.UTIL.MoveTo,MBS.UTIL.InputDiscreteArraySizem1) LIM(0,MBS.UTIL.MoveFrom,MBS.UTIL.InputDiscreteArraySizem1) [XIC(MBS.UTIL.CoilBuffer.Data[MBS.UTIL.MoveFrom]) OTL(MBS.DATA.InputBit[MBS.UTIL.MoveTo]) ,XIO(MBS.UTIL.CoilBuffer.Data[MBS.UTIL.MoveFrom]) OTU(MBS.DATA.InputBit[MBS.UTIL.MoveTo]) ] ,EQU(MBS.UTIL.Function,15) XIC(MBS.UTIL.MasterTXQuery) LIM(0,MBS.UTIL.MoveTo,MBS.UTIL.OutputDiscreteArraySizem1) LIM(0,MBS.UTIL.MoveFrom,MBS.UTIL.OutputDiscreteArraySizem1) [XIC(MBS.DATA.OutputBit[MBS.UTIL.MoveFrom]) OTL(MBS.UTIL.CoilBuffer.Data[MBS.UTIL.MoveTo]) ,XIO(MBS.DATA.OutputBit[MBS.UTIL.MoveFrom]) OTU(MBS.UTIL.CoilBuffer.Data[MBS.UTIL.MoveTo]) ] ] ,XIC(Connection_Config[5].0) [LIM(1,MBS.UTIL.Function,2) LIM(0,MBS.UTIL.MoveTo,MBS.UTIL.OutputDiscreteArraySizem1) LIM(0,MBS.UTIL.MoveFrom,MBS.UTIL.OutputDiscreteArraySizem1) [XIC(MBS.DATA.OutputBit[MBS.UTIL.MoveFrom]) OTL(MBS.UTIL.CoilBuffer.Data[MBS.UTIL.MoveTo]) ,XIO(MBS.DATA.OutputBit[MBS.UTIL.MoveFrom]) OTU(MBS.UTIL.CoilBuffer.Data[MBS.UTIL.MoveTo]) ] ,EQU(MBS.UTIL.Function,15) LIM(0,MBS.UTIL.MoveTo,MBS.UTIL.InputDiscreteArraySizem1) LIM(0,MBS.UTIL.MoveFrom,MBS.UTIL.InputDiscreteArraySizem1) [XIC(MBS.UTIL.CoilBuffer.Data[MBS.UTIL.MoveFrom]) OTL(MBS.DATA.InputBit[MBS.UTIL.MoveTo]) ,XIO(MBS.UTIL.CoilBuffer.Data[MBS.UTIL.MoveFrom]) OTU(MBS.DATA.InputBit[MBS.UTIL.MoveTo]) ] ] ];
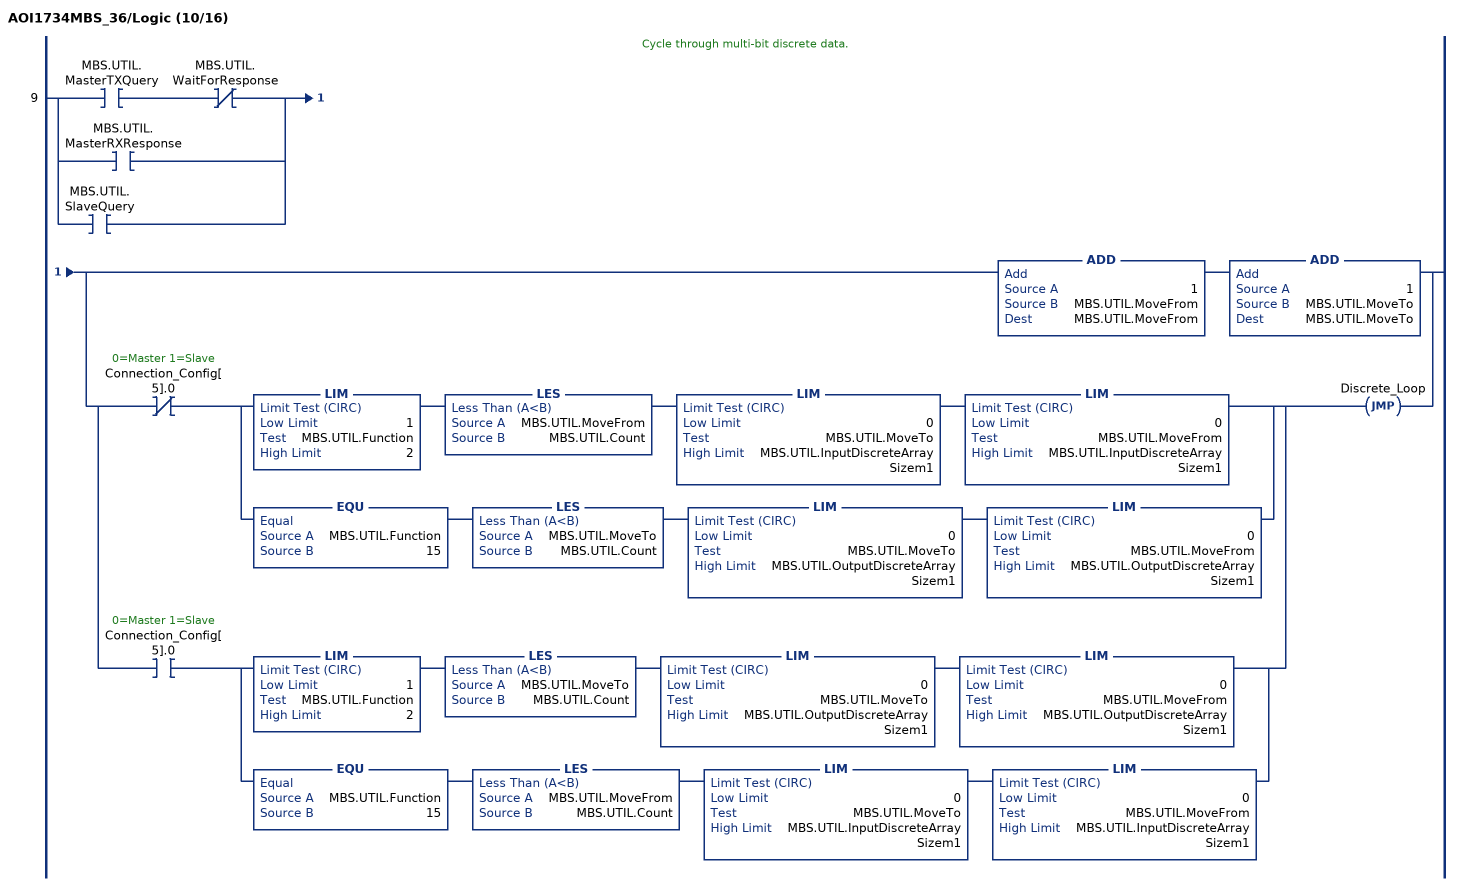
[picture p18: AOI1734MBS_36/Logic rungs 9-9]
   // Cycle through multi-bit discrete data.
   9: [XIC(MBS.UTIL.MasterTXQuery) XIO(MBS.UTIL.WaitForResponse) ,XIC(MBS.UTIL.MasterRXResponse) ,XIC(MBS.UTIL.SlaveQuery) ][ADD(1,MBS.UTIL.MoveFrom,MBS.UTIL.MoveFrom) ADD(1,MBS.UTIL.MoveTo,MBS.UTIL.MoveTo) ,[XIO(Connection_Config[5].0) [LIM(1,MBS.UTIL.Function,2) LES(MBS.UTIL.MoveFrom,MBS.UTIL.Count) LIM(0,MBS.UTIL.MoveTo,MBS.UTIL.InputDiscreteArraySizem1) LIM(0,MBS.UTIL.MoveFrom,MBS.UTIL.InputDiscreteArraySizem1) ,EQU(MBS.UTIL.Function,15) LES(MBS.UTIL.MoveTo,MBS.UTIL.Count) LIM(0,MBS.UTIL.MoveTo,MBS.UTIL.OutputDiscreteArraySizem1) LIM(0,MBS.UTIL.MoveFrom,MBS.UTIL.OutputDiscreteArraySizem1) ] ,XIC(Connection_Config[5].0) [LIM(1,MBS.UTIL.Function,2) LES(MBS.UTIL.MoveTo,MBS.UTIL.Count) LIM(0,MBS.UTIL.MoveTo,MBS.UTIL.OutputDiscreteArraySizem1) LIM(0,MBS.UTIL.MoveFrom,MBS.UTIL.OutputDiscreteArraySizem1) ,EQU(MBS.UTIL.Function,15) LES(MBS.UTIL.MoveFrom,MBS.UTIL.Count) LIM(0,MBS.UTIL.MoveTo,MBS.UTIL.InputDiscreteArraySizem1) LIM(0,MBS.UTIL.MoveFrom,MBS.UTIL.InputDiscreteArraySizem1) ] ] JMP(Discrete_Loop) ];
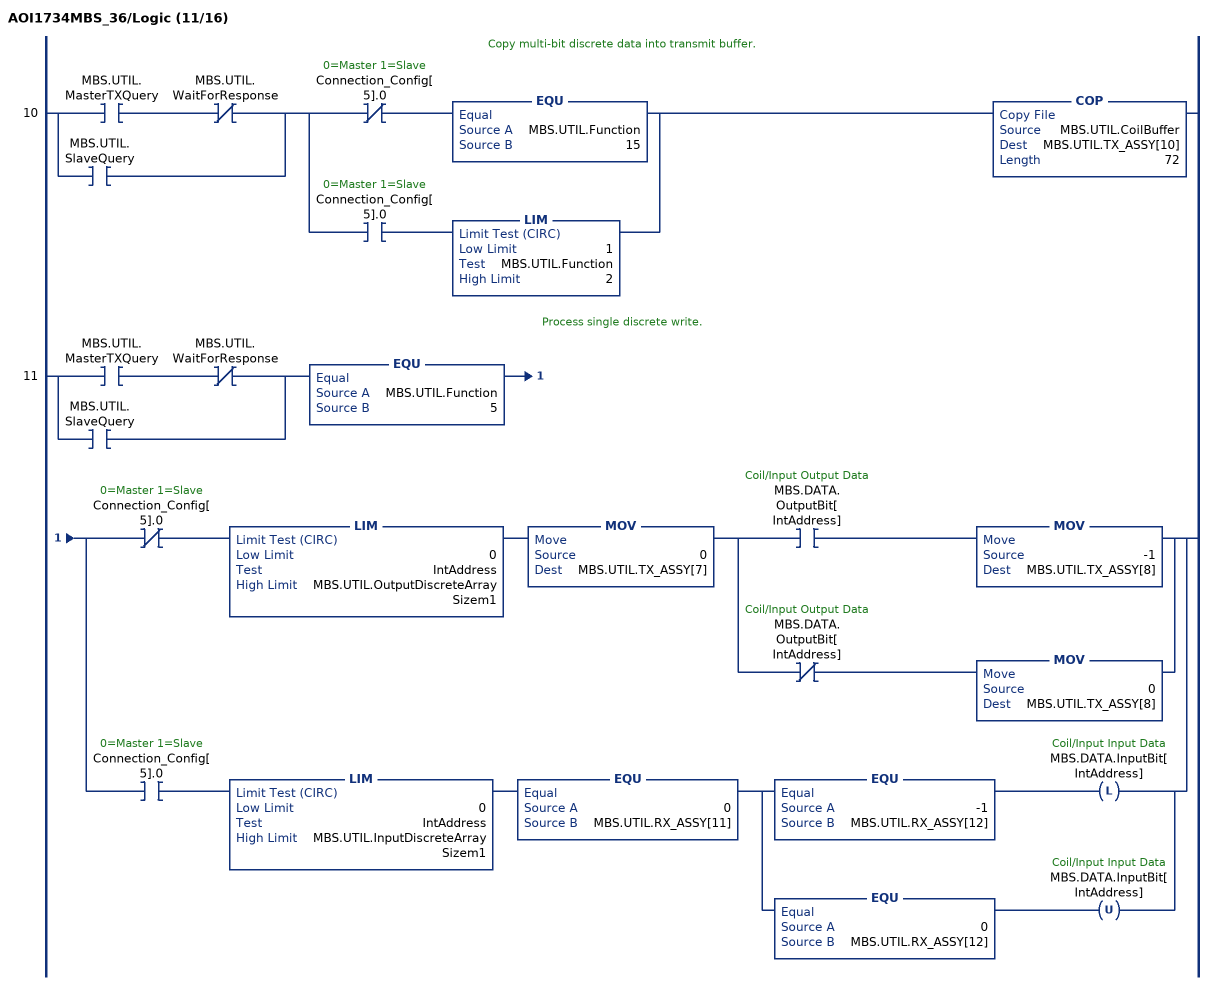
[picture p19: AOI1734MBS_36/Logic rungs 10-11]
   // Copy multi-bit discrete data into transmit buffer.
   10: [XIC(MBS.UTIL.MasterTXQuery) XIO(MBS.UTIL.WaitForResponse) ,XIC(MBS.UTIL.SlaveQuery) ][XIO(Connection_Config[5].0) EQU(MBS.UTIL.Function,15) ,XIC(Connection_Config[5].0) LIM(1,MBS.UTIL.Function,2) ]COP(MBS.UTIL.CoilBuffer,MBS.UTIL.TX_ASSY[10],72);
   // Process single discrete write.
   11: [XIC(MBS.UTIL.MasterTXQuery) XIO(MBS.UTIL.WaitForResponse) ,XIC(MBS.UTIL.SlaveQuery) ]EQU(MBS.UTIL.Function,5)[XIO(Connection_Config[5].0) LIM(0,IntAddress,MBS.UTIL.OutputDiscreteArraySizem1) MOV(0,MBS.UTIL.TX_ASSY[7]) [XIC(MBS.DATA.OutputBit[IntAddress]) MOV(-1,MBS.UTIL.TX_ASSY[8]) ,XIO(MBS.DATA.OutputBit[IntAddress]) MOV(0,MBS.UTIL.TX_ASSY[8]) ] ,XIC(Connection_Config[5].0) LIM(0,IntAddress,MBS.UTIL.InputDiscreteArraySizem1) EQU(0,MBS.UTIL.RX_ASSY[11]) [EQU(-1,MBS.UTIL.RX_ASSY[12]) OTL(MBS.DATA.InputBit[IntAddress]) ,EQU(0,MBS.UTIL.RX_ASSY[12]) OTU(MBS.DATA.InputBit[IntAddress]) ] ];
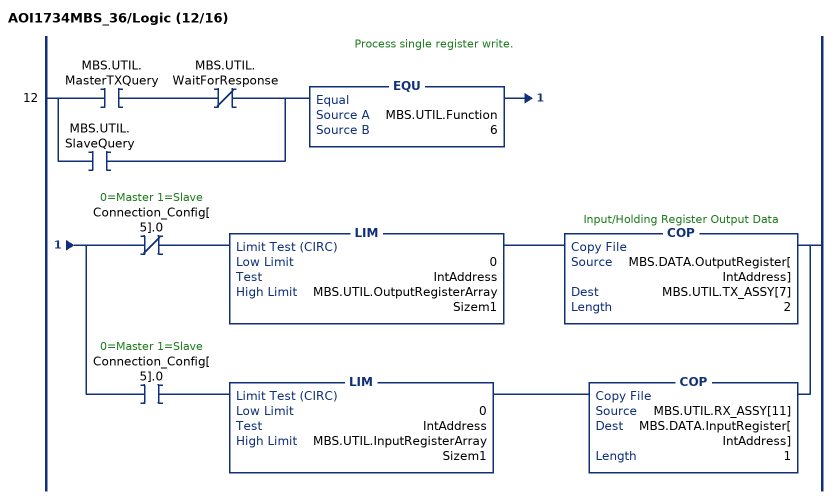
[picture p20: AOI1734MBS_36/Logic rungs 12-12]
   // Process single register write.
   12: [XIC(MBS.UTIL.MasterTXQuery) XIO(MBS.UTIL.WaitForResponse) ,XIC(MBS.UTIL.SlaveQuery) ]EQU(MBS.UTIL.Function,6)[XIO(Connection_Config[5].0) LIM(0,IntAddress,MBS.UTIL.OutputRegisterArraySizem1) COP(MBS.DATA.OutputRegister[IntAddress],MBS.UTIL.TX_ASSY[7],2) ,XIC(Connection_Config[5].0) LIM(0,IntAddress,MBS.UTIL.InputRegisterArraySizem1) COP(MBS.UTIL.RX_ASSY[11],MBS.DATA.InputRegister[IntAddress],1) ];
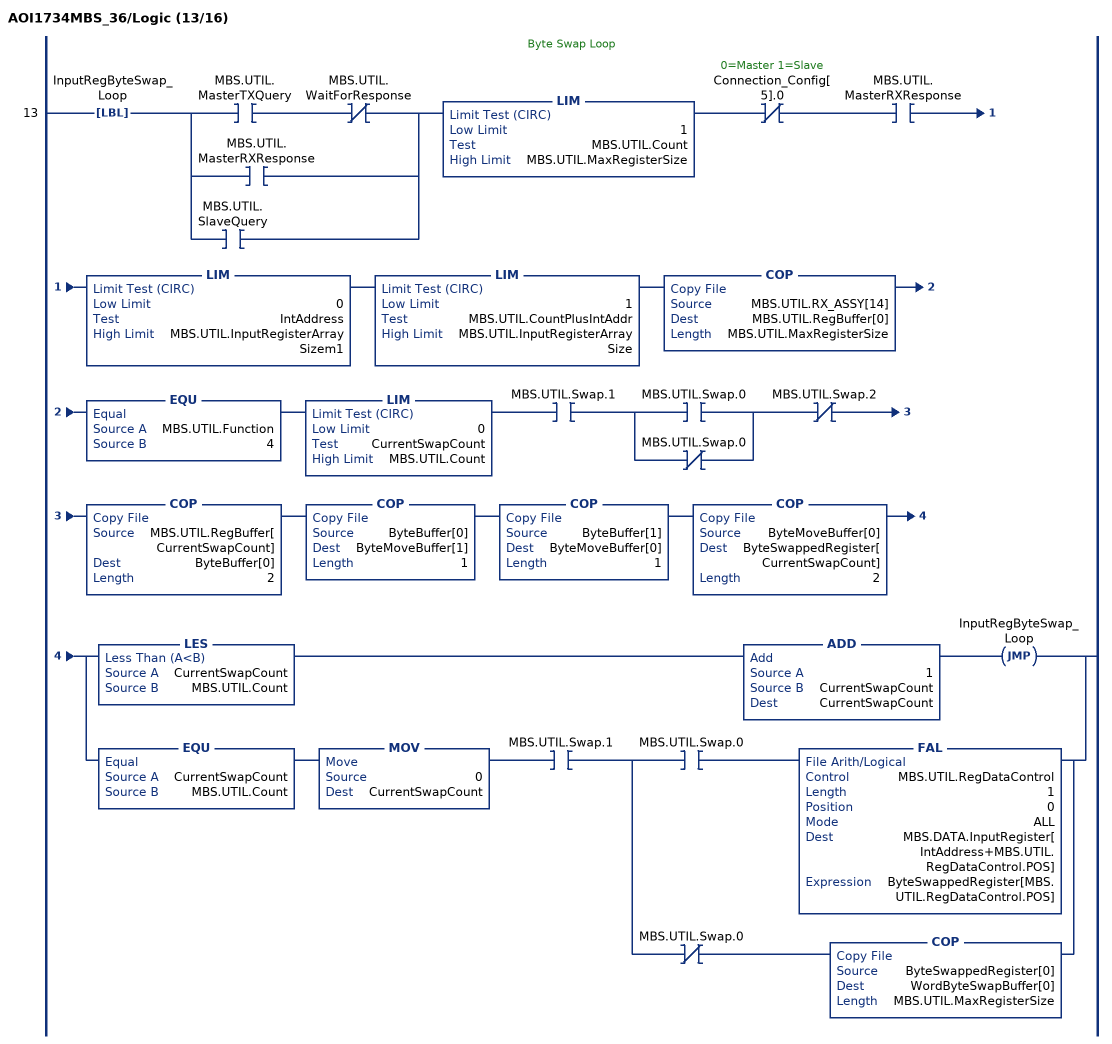
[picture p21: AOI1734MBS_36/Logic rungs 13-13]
   // Byte Swap Loop
   13: LBL(InputRegByteSwap_Loop)[XIC(MBS.UTIL.MasterTXQuery) XIO(MBS.UTIL.WaitForResponse) ,XIC(MBS.UTIL.MasterRXResponse) ,XIC(MBS.UTIL.SlaveQuery) ]LIM(1,MBS.UTIL.Count,MBS.UTIL.MaxRegisterSize)XIO(Connection_Config[5].0)XIC(MBS.UTIL.MasterRXResponse)LIM(0,IntAddress,MBS.UTIL.InputRegisterArraySizem1)LIM(1,MBS.UTIL.CountPlusIntAddr,MBS.UTIL.InputRegisterArraySize)COP(MBS.UTIL.RX_ASSY[14],MBS.UTIL.RegBuffer[0],MBS.UTIL.MaxRegisterSize)EQU(MBS.UTIL.Function,4)LIM(0,CurrentSwapCount,MBS.UTIL.Count)XIC(MBS.UTIL.Swap.1)[XIC(MBS.UTIL.Swap.0) ,XIO(MBS.UTIL.Swap.0) ]XIO(MBS.UTIL.Swap.2)COP(MBS.UTIL.RegBuffer[CurrentSwapCount],ByteBuffer[0],2)COP(ByteBuffer[0],ByteMoveBuffer[1],1)COP(ByteBuffer[1],ByteMoveBuffer[0],1)COP(ByteMoveBuffer[0],ByteSwappedRegister[CurrentSwapCount],2)[LES(CurrentSwapCount,MBS.UTIL.Count) ADD(1,CurrentSwapCount,CurrentSwapCount) JMP(InputRegByteSwap_Loop) ,EQU(CurrentSwapCount,MBS.UTIL.Count) MOV(0,CurrentSwapCount) XIC(MBS.UTIL.Swap.1) [XIC(MBS.UTIL.Swap.0) FAL(MBS.UTIL.RegDataControl,1,0,ALL,MBS.DATA.InputRegister[IntAddress+MBS.UTIL.RegDataControl.POS],ByteSwappedRegister[MBS.UTIL.RegDataControl.POS]) ,XIO(MBS.UTIL.Swap.0) COP(ByteSwappedRegister[0],WordByteSwapBuffer[0],MBS.UTIL.MaxRegisterSize) ] ];
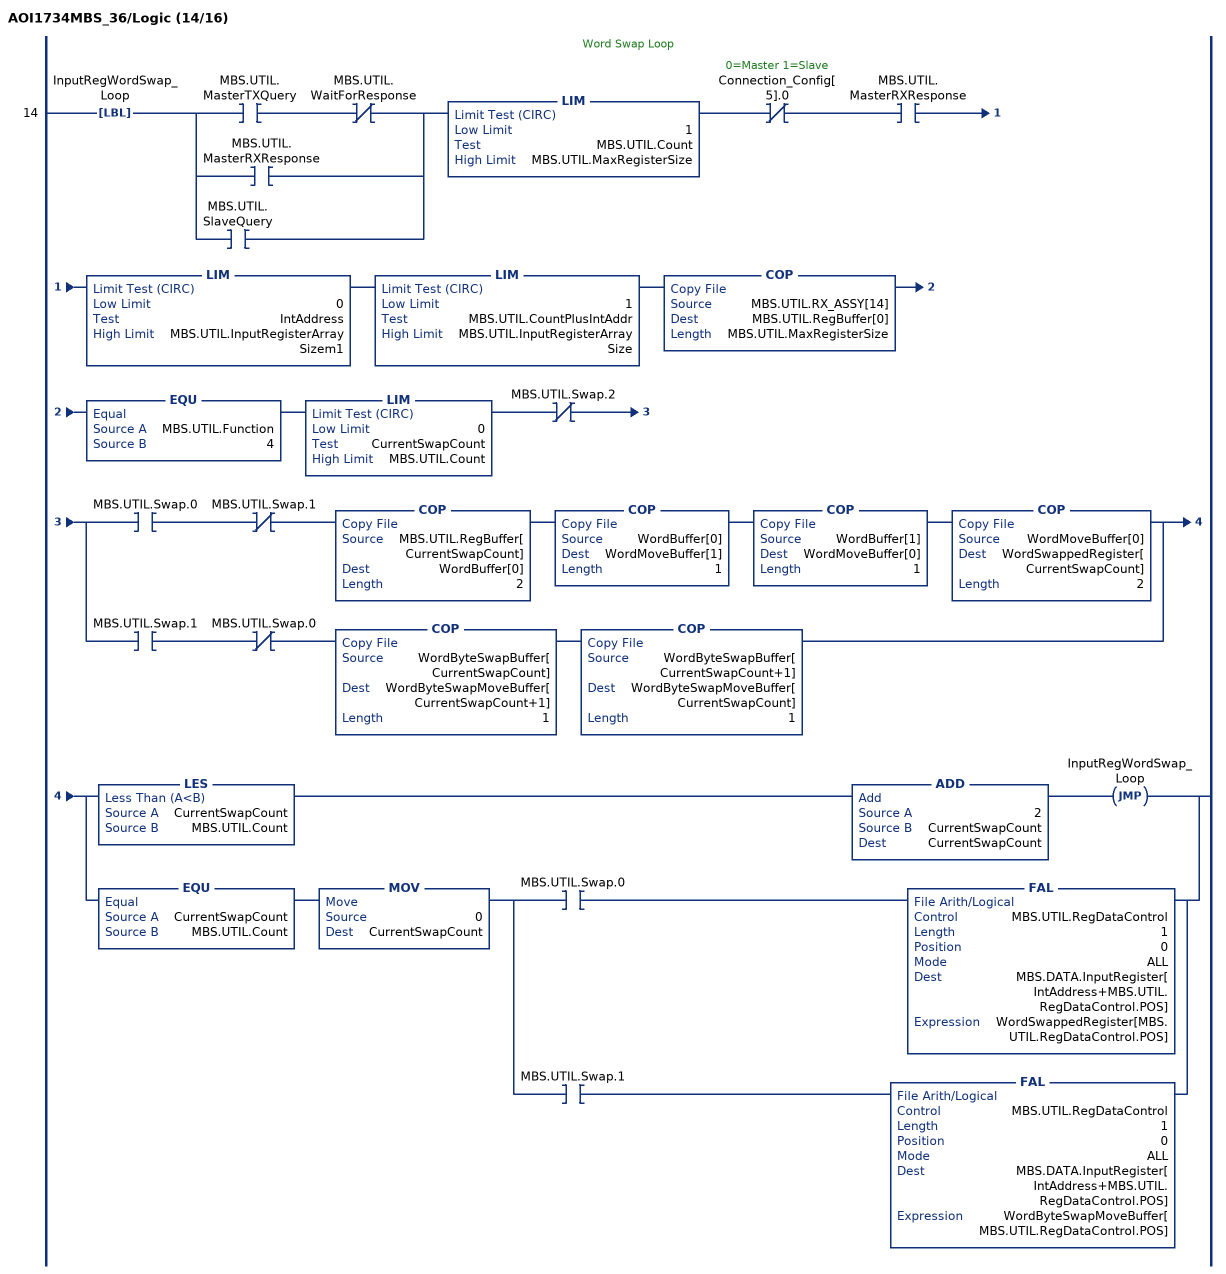
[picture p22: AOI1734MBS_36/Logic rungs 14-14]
   // Word Swap Loop
   14: LBL(InputRegWordSwap_Loop)[XIC(MBS.UTIL.MasterTXQuery) XIO(MBS.UTIL.WaitForResponse) ,XIC(MBS.UTIL.MasterRXResponse) ,XIC(MBS.UTIL.SlaveQuery) ]LIM(1,MBS.UTIL.Count,MBS.UTIL.MaxRegisterSize)XIO(Connection_Config[5].0)XIC(MBS.UTIL.MasterRXResponse)LIM(0,IntAddress,MBS.UTIL.InputRegisterArraySizem1)LIM(1,MBS.UTIL.CountPlusIntAddr,MBS.UTIL.InputRegisterArraySize)COP(MBS.UTIL.RX_ASSY[14],MBS.UTIL.RegBuffer[0],MBS.UTIL.MaxRegisterSize)EQU(MBS.UTIL.Function,4)LIM(0,CurrentSwapCount,MBS.UTIL.Count)XIO(MBS.UTIL.Swap.2)[XIC(MBS.UTIL.Swap.0) XIO(MBS.UTIL.Swap.1) COP(MBS.UTIL.RegBuffer[CurrentSwapCount],WordBuffer[0],2) COP(WordBuffer[0],WordMoveBuffer[1],1) COP(WordBuffer[1],WordMoveBuffer[0],1) COP(WordMoveBuffer[0],WordSwappedRegister[CurrentSwapCount],2) ,XIC(MBS.UTIL.Swap.1) XIO(MBS.UTIL.Swap.0) COP(WordByteSwapBuffer[CurrentSwapCount],WordByteSwapMoveBuffer[CurrentSwapCount+1],1) COP(WordByteSwapBuffer[CurrentSwapCount+1],WordByteSwapMoveBuffer[CurrentSwapCount],1) ][LES(CurrentSwapCount,MBS.UTIL.Count) ADD(2,CurrentSwapCount,CurrentSwapCount) JMP(InputRegWordSwap_Loop) ,EQU(CurrentSwapCount,MBS.UTIL.Count) MOV(0,CurrentSwapCount) [XIC(MBS.UTIL.Swap.0) FAL(MBS.UTIL.RegDataControl,1,0,ALL,MBS.DATA.InputRegister[IntAddress+MBS.UTIL.RegDataControl.POS],WordSwappedRegister[MBS.UTIL.RegDataControl.POS]) ,XIC(MBS.UTIL.Swap.1) FAL(MBS.UTIL.RegDataControl,1,0,ALL,MBS.DATA.InputRegister[IntAddress+MBS.UTIL.RegDataControl.POS],WordByteSwapMoveBuffer[MBS.UTIL.RegDataControl.POS]) ] ];
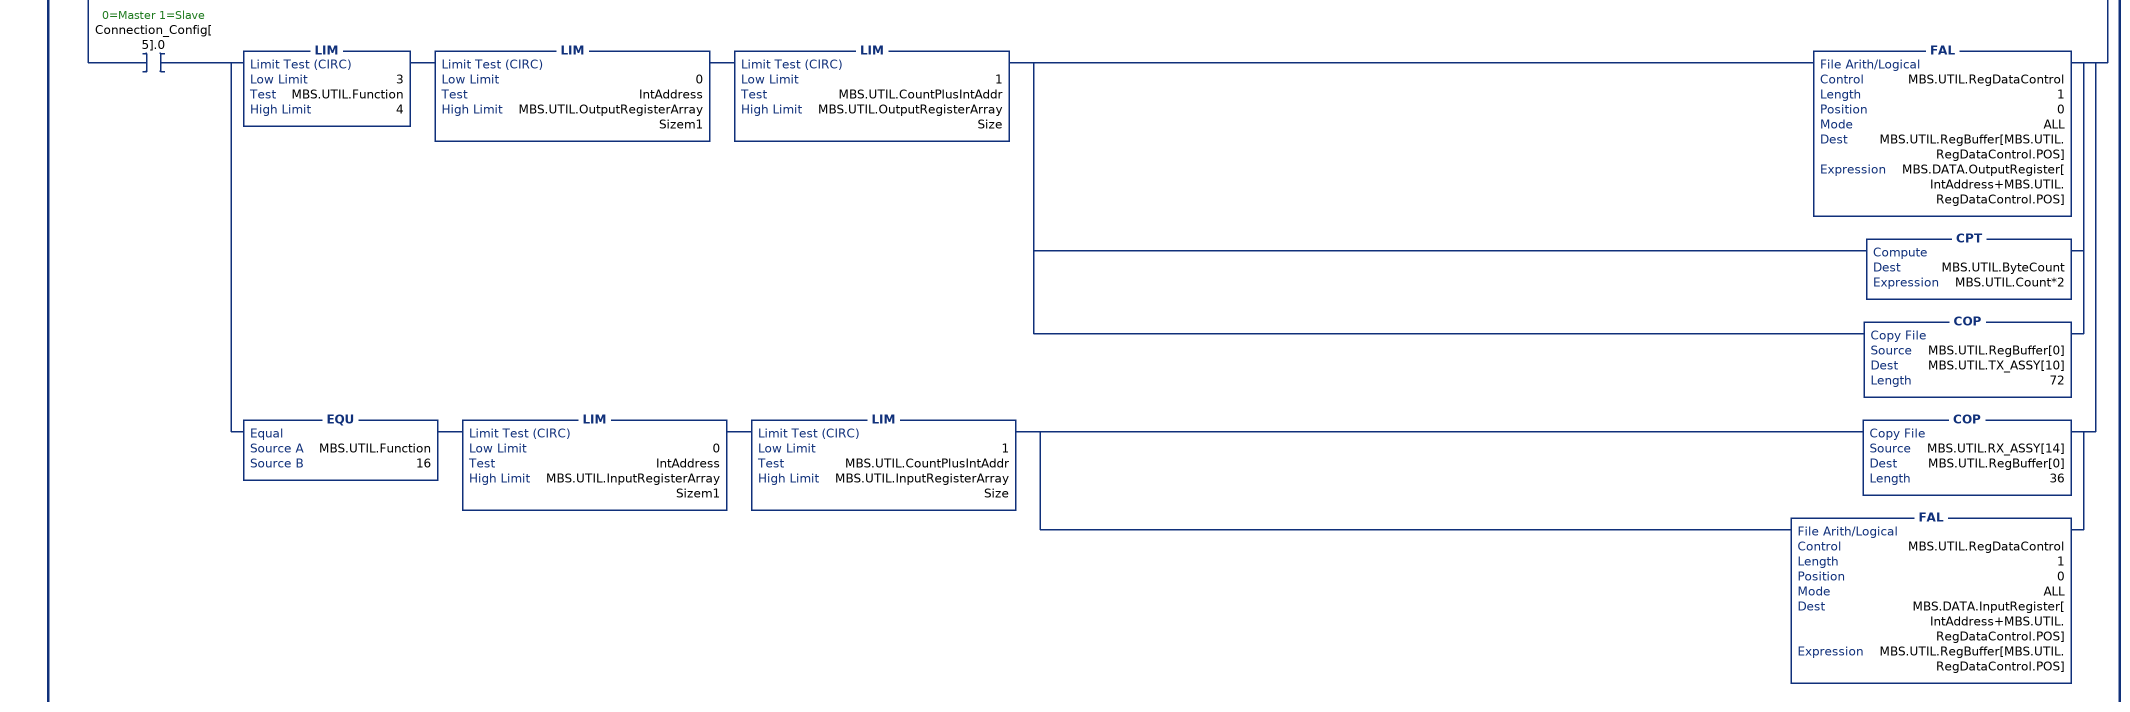
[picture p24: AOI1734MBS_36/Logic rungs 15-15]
   // Process multi-register functions.
   15: [XIC(MBS.UTIL.MasterTXQuery) XIO(MBS.UTIL.WaitForResponse) ,XIC(MBS.UTIL.MasterRXResponse) ,XIC(MBS.UTIL.SlaveQuery) ]LIM(1,MBS.UTIL.Count,MBS.UTIL.MaxRegisterSize)[MOV(MBS.UTIL.Count,MBS.UTIL.RegDataControl.LEN) MOV(0,MBS.UTIL.RegDataControl.POS) OTU(MBS.UTIL.RegDataControl.ER) OTU(MBS.UTIL.RegDataControl.DN) ,[XIO(Connection_Config[5].0) [XIC(MBS.UTIL.MasterRXResponse) LIM(3,MBS.UTIL.Function,4) LIM(0,IntAddress,MBS.UTIL.InputRegisterArraySizem1) LIM(1,MBS.UTIL.CountPlusIntAddr,MBS.UTIL.InputRegisterArraySize) [COP(MBS.UTIL.RX_ASSY[14],MBS.UTIL.RegBuffer[0],MBS.UTIL.MaxRegisterSize) ,[EQU(MBS.UTIL.Function,3) ,EQU(MBS.UTIL.Function,4) XIO(MBS.UTIL.Swap.0) XIO(MBS.UTIL.Swap.1) XIO(MBS.UTIL.Swap.2) ] FAL(MBS.UTIL.RegDataControl,1,0,ALL,MBS.DATA.InputRegister[IntAddress+MBS.UTIL.RegDataControl.POS],MBS.UTIL.RegBuffer[MBS.UTIL.RegDataControl.POS]) ] ,XIC(MBS.UTIL.MasterTXQuery) EQU(MBS.UTIL.Function,16) LIM(0,IntAddress,MBS.UTIL.OutputRegisterArraySizem1) LIM(1,MBS.UTIL.CountPlusIntAddr,MBS.UTIL.OutputRegisterArraySize) [FAL(MBS.UTIL.RegDataControl,1,0,ALL,MBS.UTIL.RegBuffer[MBS.UTIL.RegDataControl.POS],MBS.DATA.OutputRegister[IntAddress+MBS.UTIL.RegDataControl.POS]) ,CPT(MBS.UTIL.ByteCount,MBS.UTIL.Count*2) ,COP(MBS.UTIL.RegBuffer[0],MBS.UTIL.TX_ASSY[10],72) ] ] ,XIC(Connection_Config[5].0) [LIM(3,MBS.UTIL.Function,4) LIM(0,IntAddress,MBS.UTIL.OutputRegisterArraySizem1) LIM(1,MBS.UTIL.CountPlusIntAddr,MBS.UTIL.OutputRegisterArraySize) [FAL(MBS.UTIL.RegDataControl,1,0,ALL,MBS.UTIL.RegBuffer[MBS.UTIL.RegDataControl.POS],MBS.DATA.OutputRegister[IntAddress+MBS.UTIL.RegDataControl.POS]) ,CPT(MBS.UTIL.ByteCount,MBS.UTIL.Count*2) ,COP(MBS.UTIL.RegBuffer[0],MBS.UTIL.TX_ASSY[10],72) ] ,EQU(MBS.UTIL.Function,16) LIM(0,IntAddress,MBS.UTIL.InputRegisterArraySizem1) LIM(1,MBS.UTIL.CountPlusIntAddr,MBS.UTIL.InputRegisterArraySize) [COP(MBS.UTIL.RX_ASSY[14],MBS.UTIL.RegBuffer[0],36) ,FAL(MBS.UTIL.RegDataControl,1,0,ALL,MBS.DATA.InputRegister[IntAddress+MBS.UTIL.RegDataControl.POS],MBS.UTIL.RegBuffer[MBS.UTIL.RegDataControl.POS]) ] ] ] ];
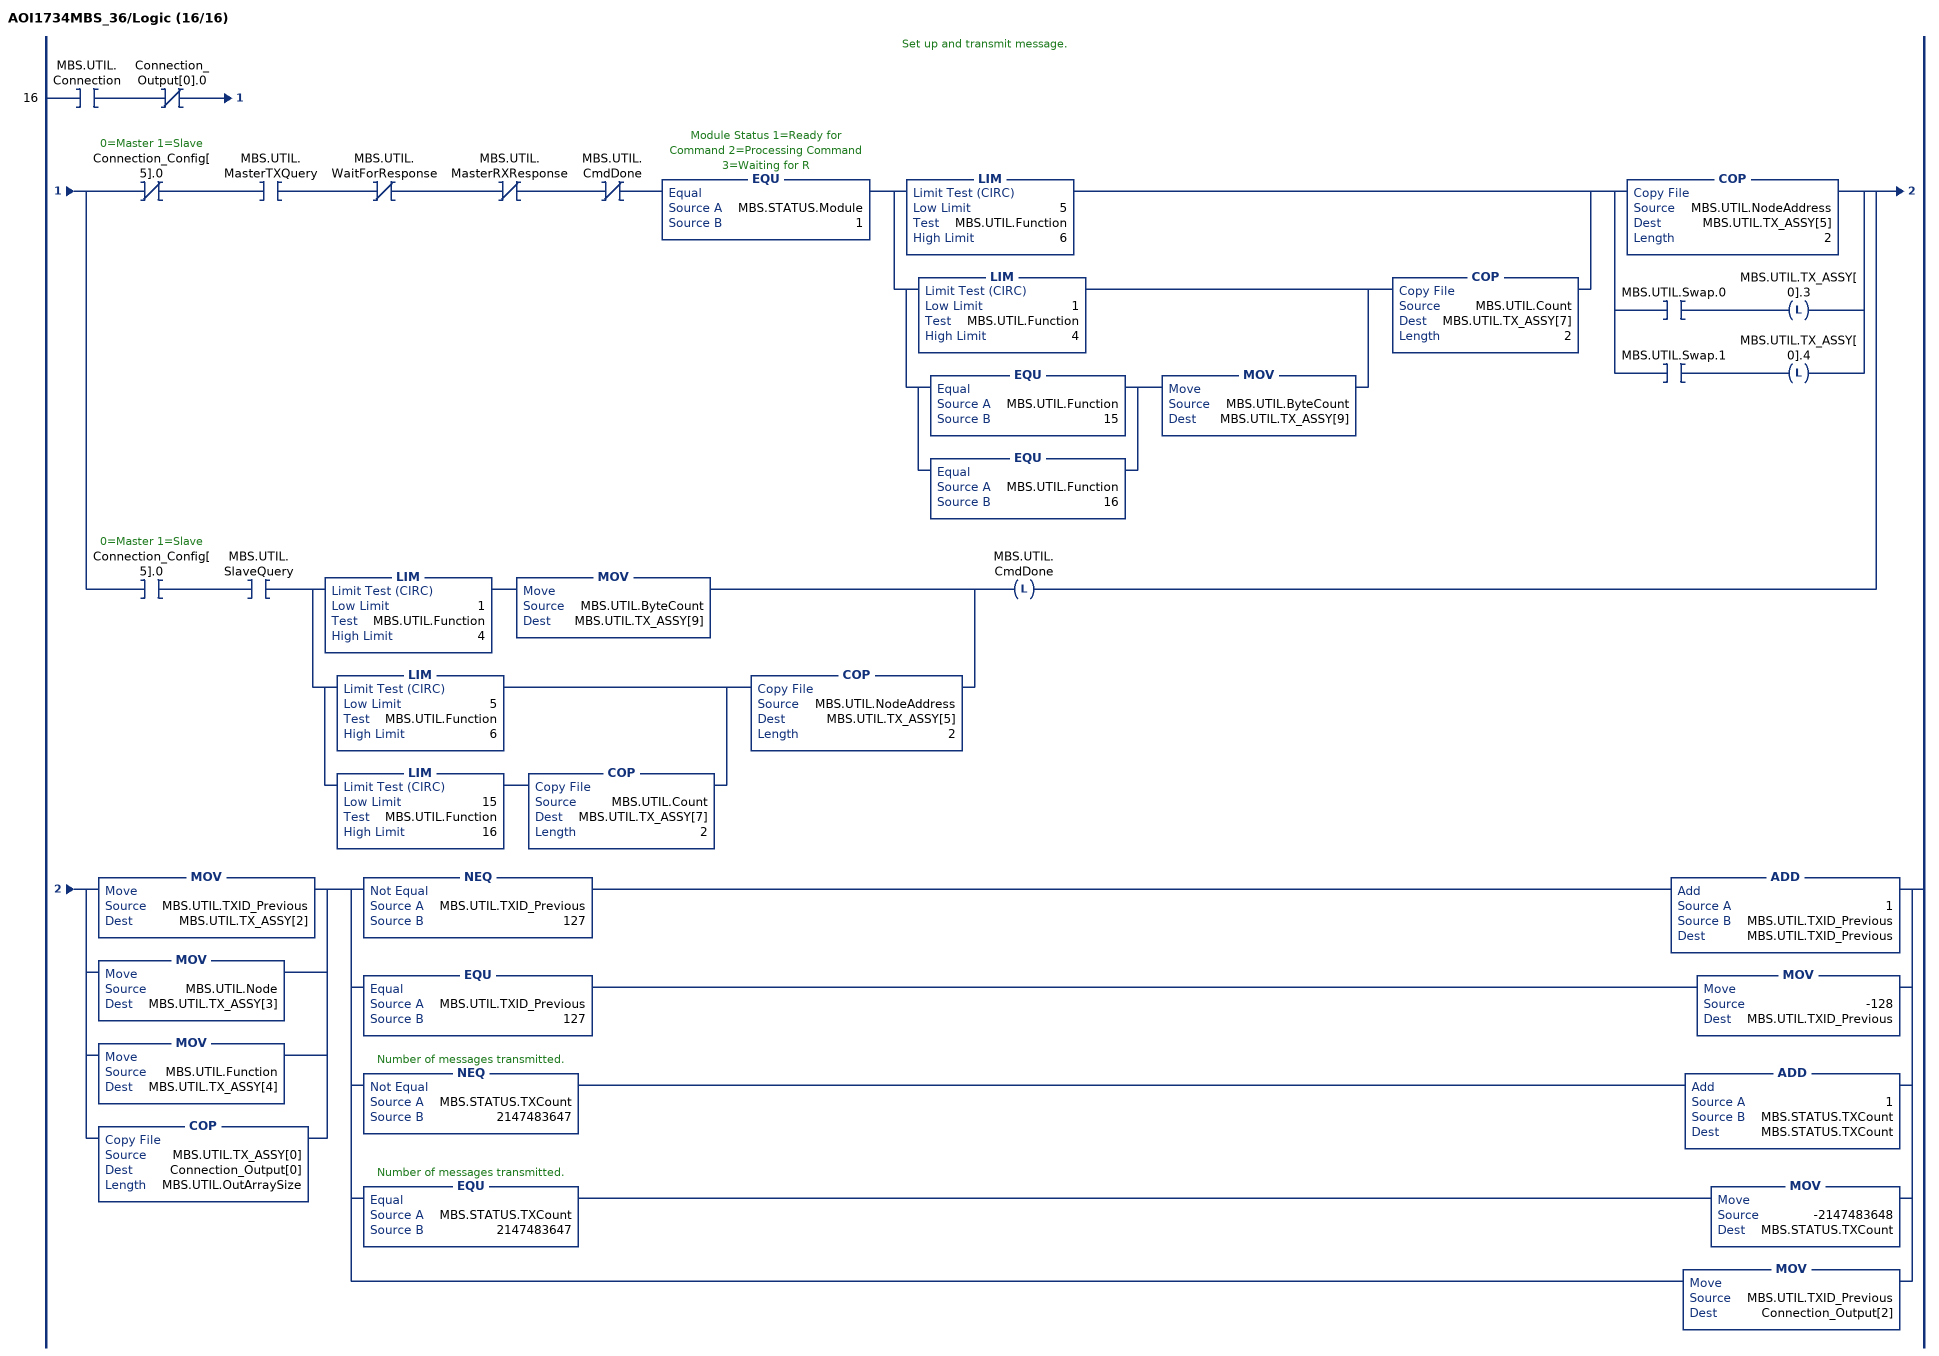
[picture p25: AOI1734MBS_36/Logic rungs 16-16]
   // Set up and transmit message.
   16: XIC(MBS.UTIL.Connection)XIO(Connection_Output[0].0)[XIO(Connection_Config[5].0) XIC(MBS.UTIL.MasterTXQuery) XIO(MBS.UTIL.WaitForResponse) XIO(MBS.UTIL.MasterRXResponse) XIO(MBS.UTIL.CmdDone) EQU(MBS.STATUS.Module,1) [LIM(5,MBS.UTIL.Function,6) ,[LIM(1,MBS.UTIL.Function,4) ,[EQU(MBS.UTIL.Function,15) ,EQU(MBS.UTIL.Function,16) ] MOV(MBS.UTIL.ByteCount,MBS.UTIL.TX_ASSY[9]) ] COP(MBS.UTIL.Count,MBS.UTIL.TX_ASSY[7],2) ] [COP(MBS.UTIL.NodeAddress,MBS.UTIL.TX_ASSY[5],2) ,XIC(MBS.UTIL.Swap.0) OTL(MBS.UTIL.TX_ASSY[0].3) ,XIC(MBS.UTIL.Swap.1) OTL(MBS.UTIL.TX_ASSY[0].4) ] ,XIC(Connection_Config[5].0) XIC(MBS.UTIL.SlaveQuery) [LIM(1,MBS.UTIL.Function,4) MOV(MBS.UTIL.ByteCount,MBS.UTIL.TX_ASSY[9]) ,[LIM(5,MBS.UTIL.Function,6) ,LIM(15,MBS.UTIL.Function,16) COP(MBS.UTIL.Count,MBS.UTIL.TX_ASSY[7],2) ] COP(MBS.UTIL.NodeAddress,MBS.UTIL.TX_ASSY[5],2) ] OTL(MBS.UTIL.CmdDone) ][MOV(MBS.UTIL.TXID_Previous,MBS.UTIL.TX_ASSY[2]) ,MOV(MBS.UTIL.Node,MBS.UTIL.TX_ASSY[3]) ,MOV(MBS.UTIL.Function,MBS.UTIL.TX_ASSY[4]) ,COP(MBS.UTIL.TX_ASSY[0],Connection_Output[0],MBS.UTIL.OutArraySize) ][[NEQ(MBS.UTIL.TXID_Previous,127) ADD(1,MBS.UTIL.TXID_Previous,MBS.UTIL.TXID_Previous) ,EQU(MBS.UTIL.TXID_Previous,127) MOV(-128,MBS.UTIL.TXID_Previous) ] ,[NEQ(MBS.STATUS.TXCount,2147483647) ADD(1,MBS.STATUS.TXCount,MBS.STATUS.TXCount) ,EQU(MBS.STATUS.TXCount,2147483647) MOV(-2147483648,MBS.STATUS.TXCount) ] ,MOV(MBS.UTIL.TXID_Previous,Connection_Output[2]) ];
END_ROUTINE

ROUTINE Prescan   (* ladder *)
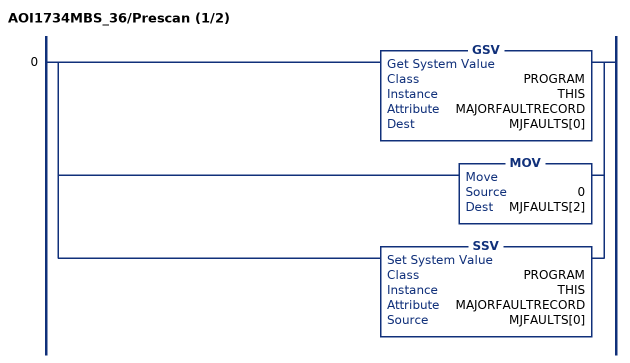
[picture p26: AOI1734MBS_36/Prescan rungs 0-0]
   0: [GSV(PROGRAM,THIS,MAJORFAULTRECORD,MJFAULTS[0]) ,MOV(0,MJFAULTS[2]) ,SSV(PROGRAM,THIS,MAJORFAULTRECORD,MJFAULTS[0]) ];
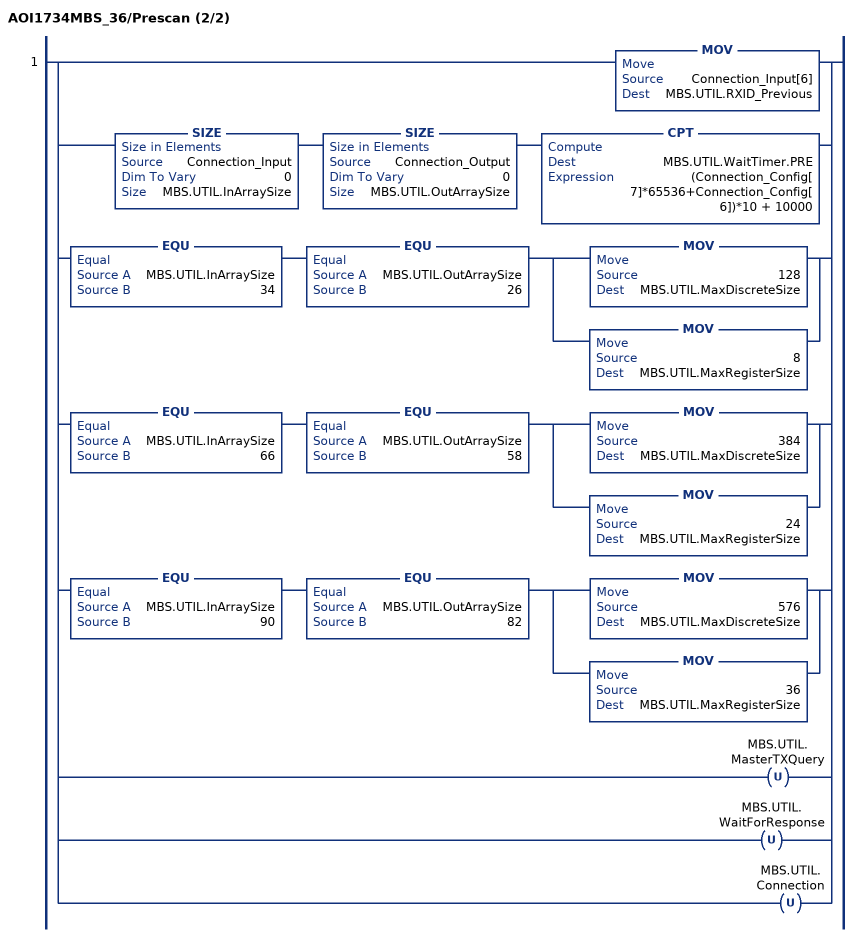
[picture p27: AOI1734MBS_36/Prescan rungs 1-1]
   1: [MOV(Connection_Input[6],MBS.UTIL.RXID_Previous) ,SIZE(Connection_Input,0,MBS.UTIL.InArraySize) SIZE(Connection_Output,0,MBS.UTIL.OutArraySize) CPT(MBS.UTIL.WaitTimer.PRE,(Connection_Config[7]*65536+Connection_Config[6])*10 + 10000) ,EQU(MBS.UTIL.InArraySize,34) EQU(MBS.UTIL.OutArraySize,26) [MOV(128,MBS.UTIL.MaxDiscreteSize) ,MOV(8,MBS.UTIL.MaxRegisterSize) ] ,EQU(MBS.UTIL.InArraySize,66) EQU(MBS.UTIL.OutArraySize,58) [MOV(384,MBS.UTIL.MaxDiscreteSize) ,MOV(24,MBS.UTIL.MaxRegisterSize) ] ,EQU(MBS.UTIL.InArraySize,90) EQU(MBS.UTIL.OutArraySize,82) [MOV(576,MBS.UTIL.MaxDiscreteSize) ,MOV(36,MBS.UTIL.MaxRegisterSize) ] ,OTU(MBS.UTIL.MasterTXQuery) ,OTU(MBS.UTIL.WaitForResponse) ,OTU(MBS.UTIL.Connection) ];
END_ROUTINE
END_ADD_ON_INSTRUCTION
